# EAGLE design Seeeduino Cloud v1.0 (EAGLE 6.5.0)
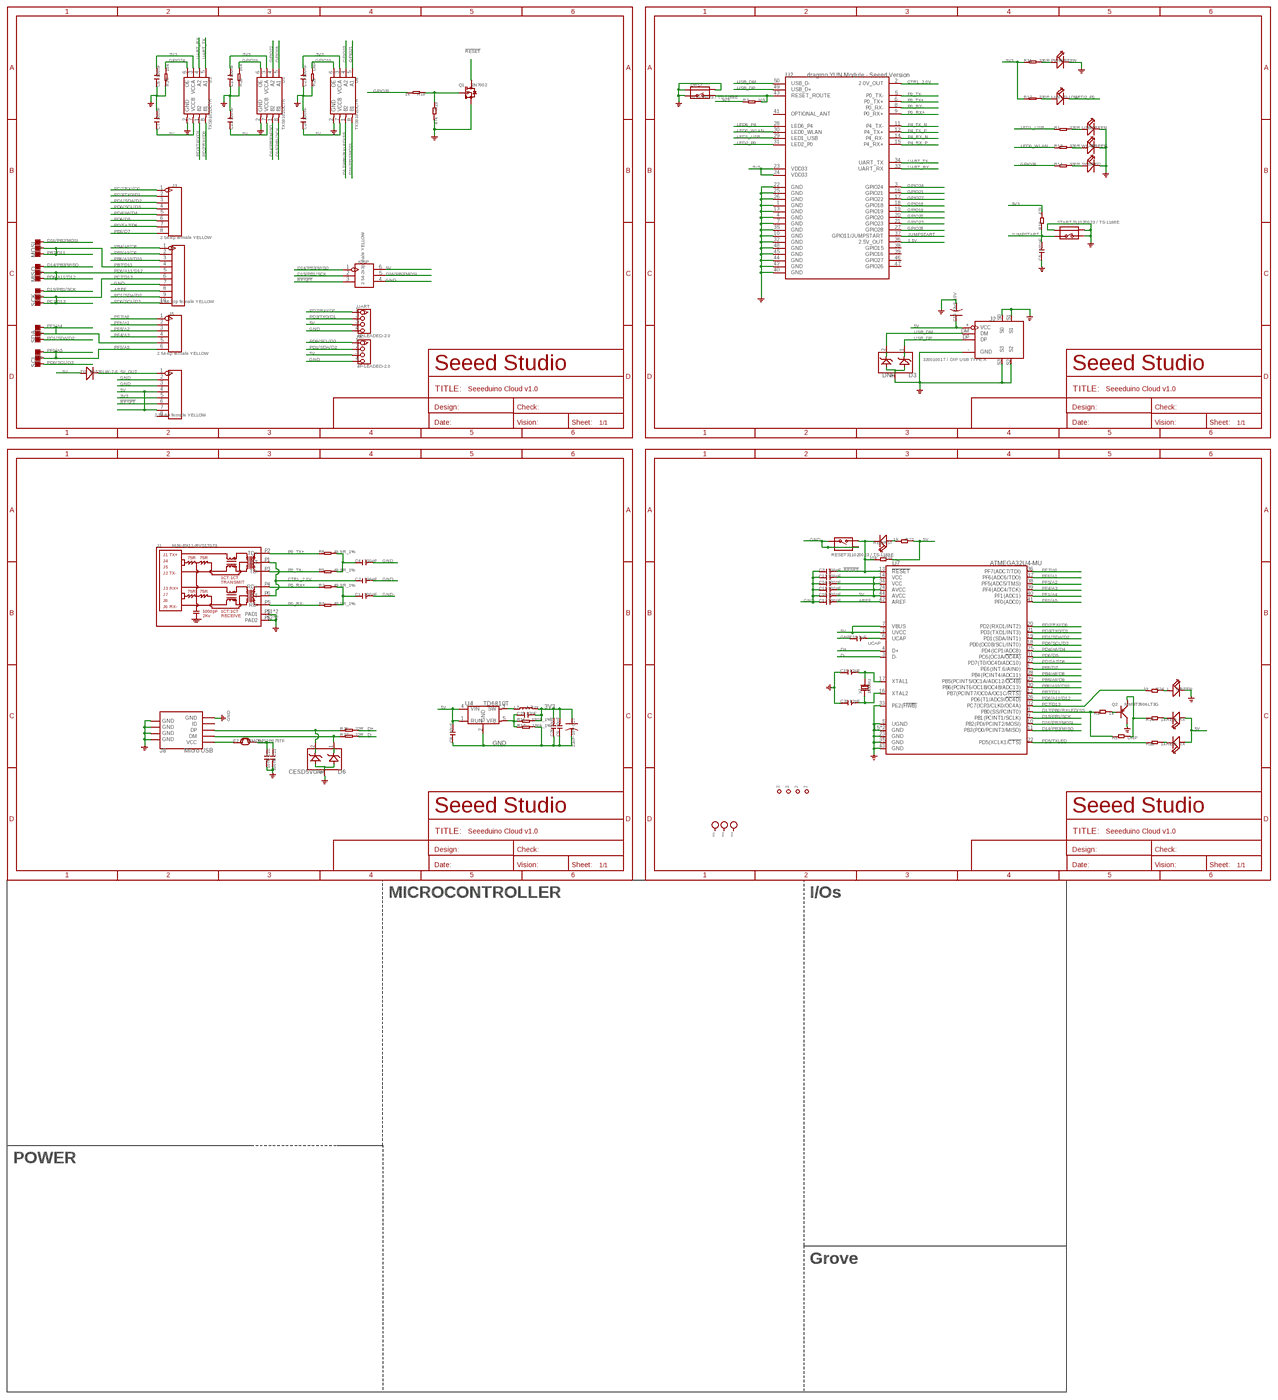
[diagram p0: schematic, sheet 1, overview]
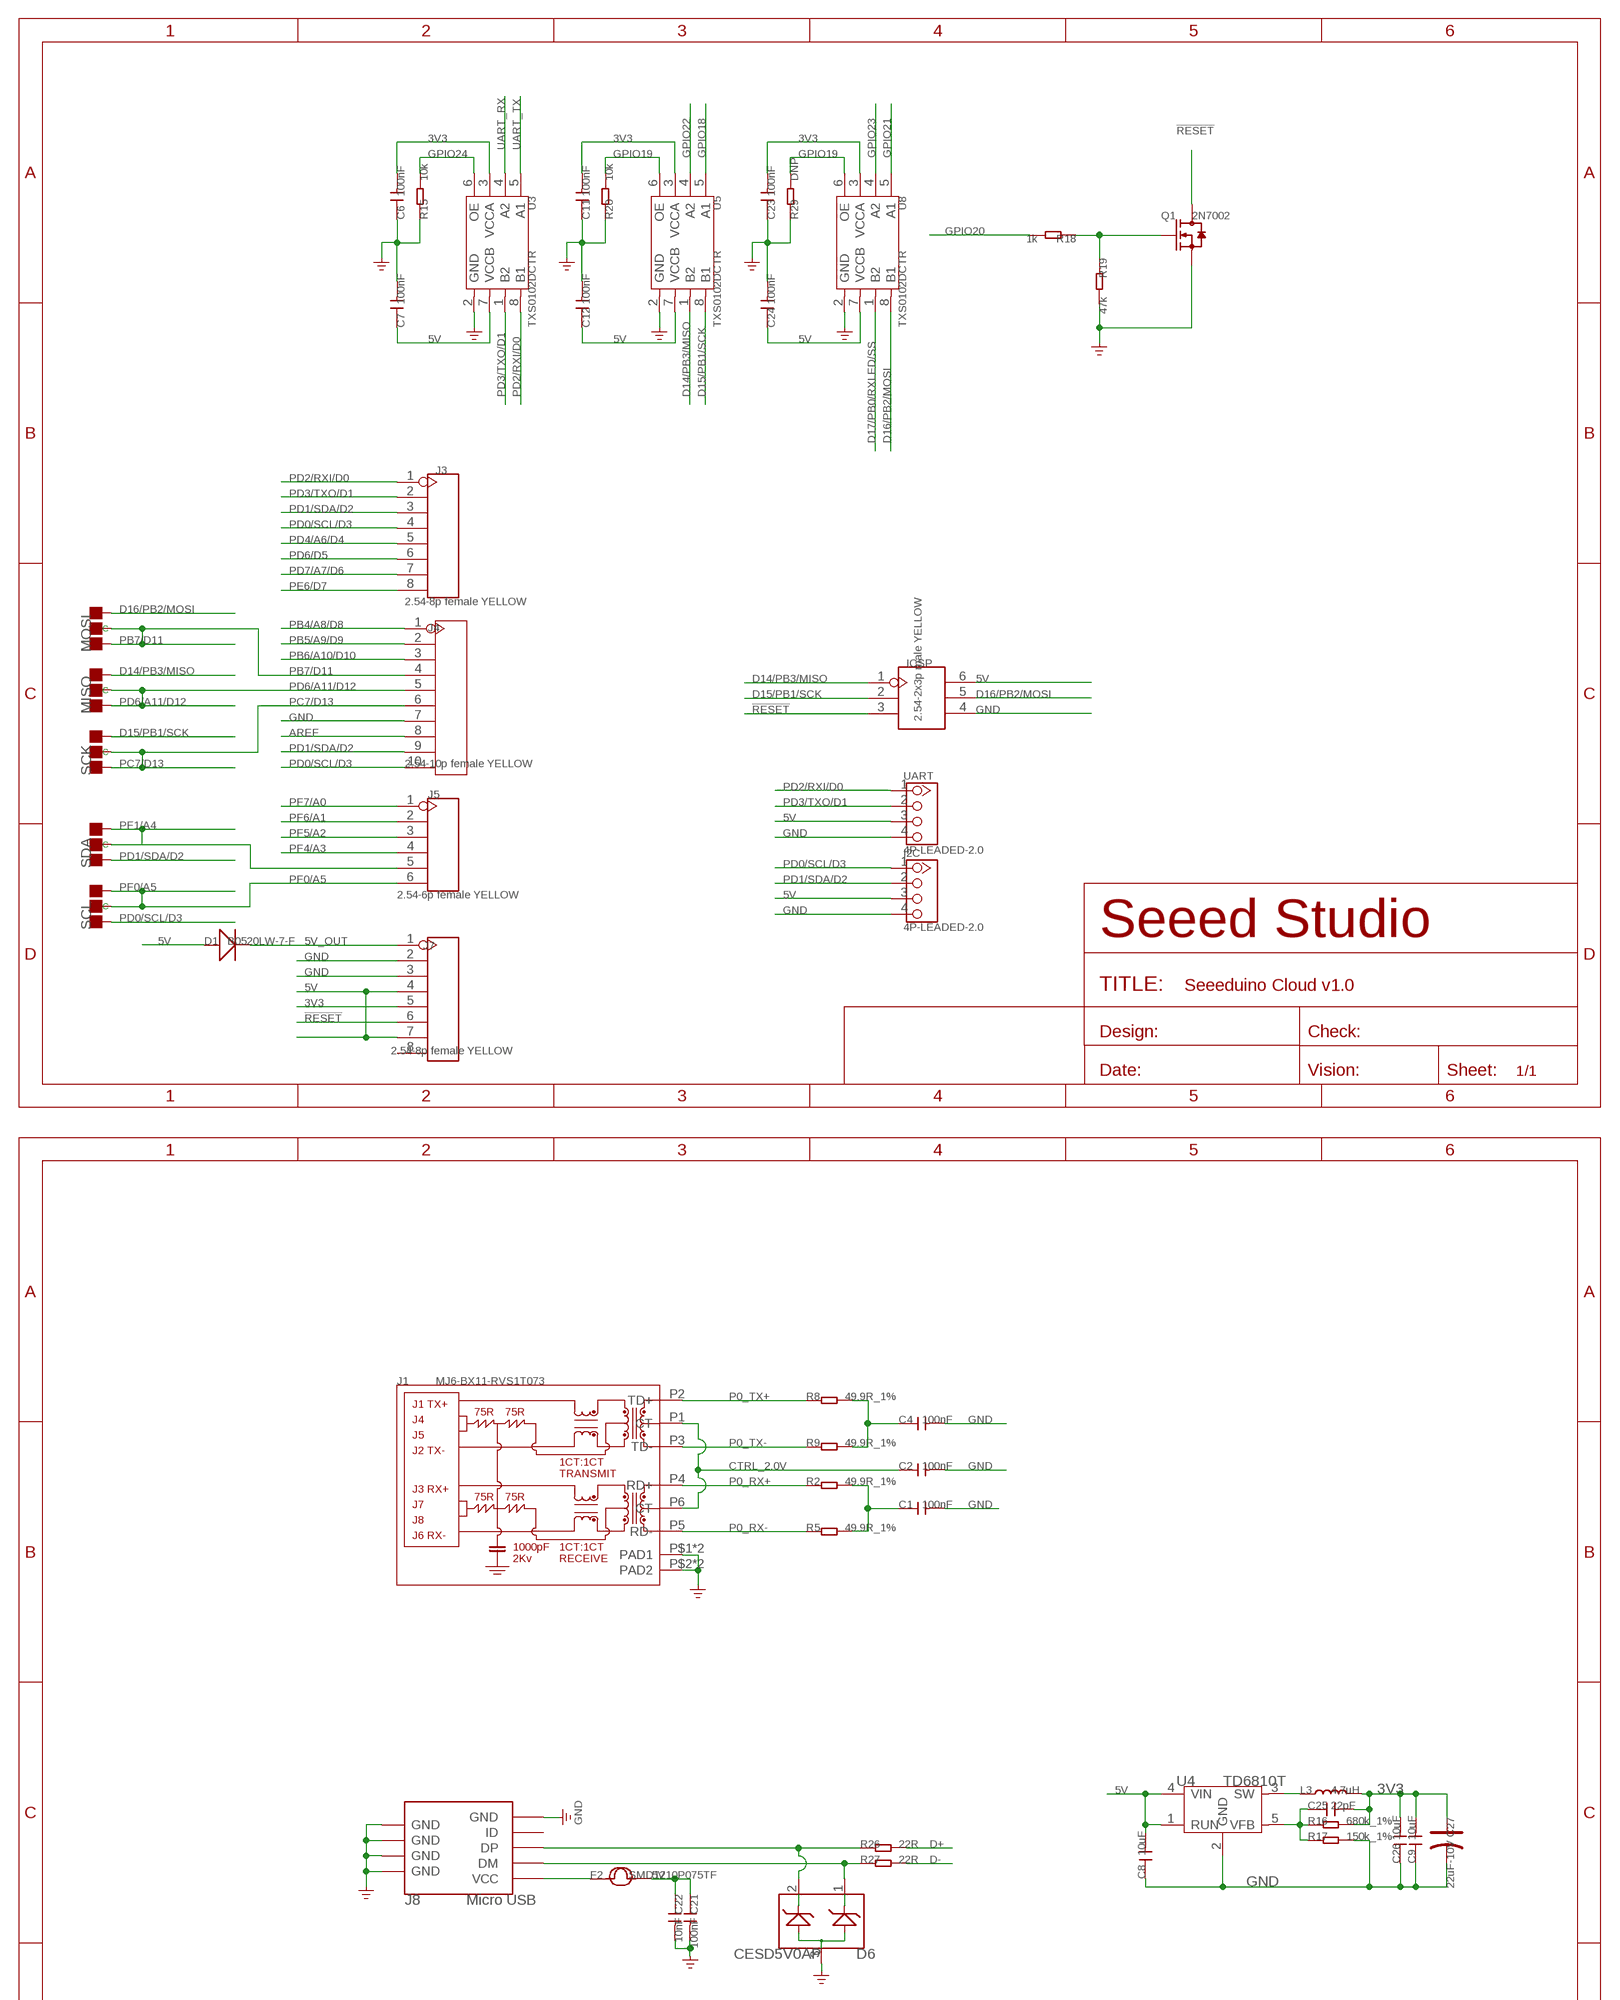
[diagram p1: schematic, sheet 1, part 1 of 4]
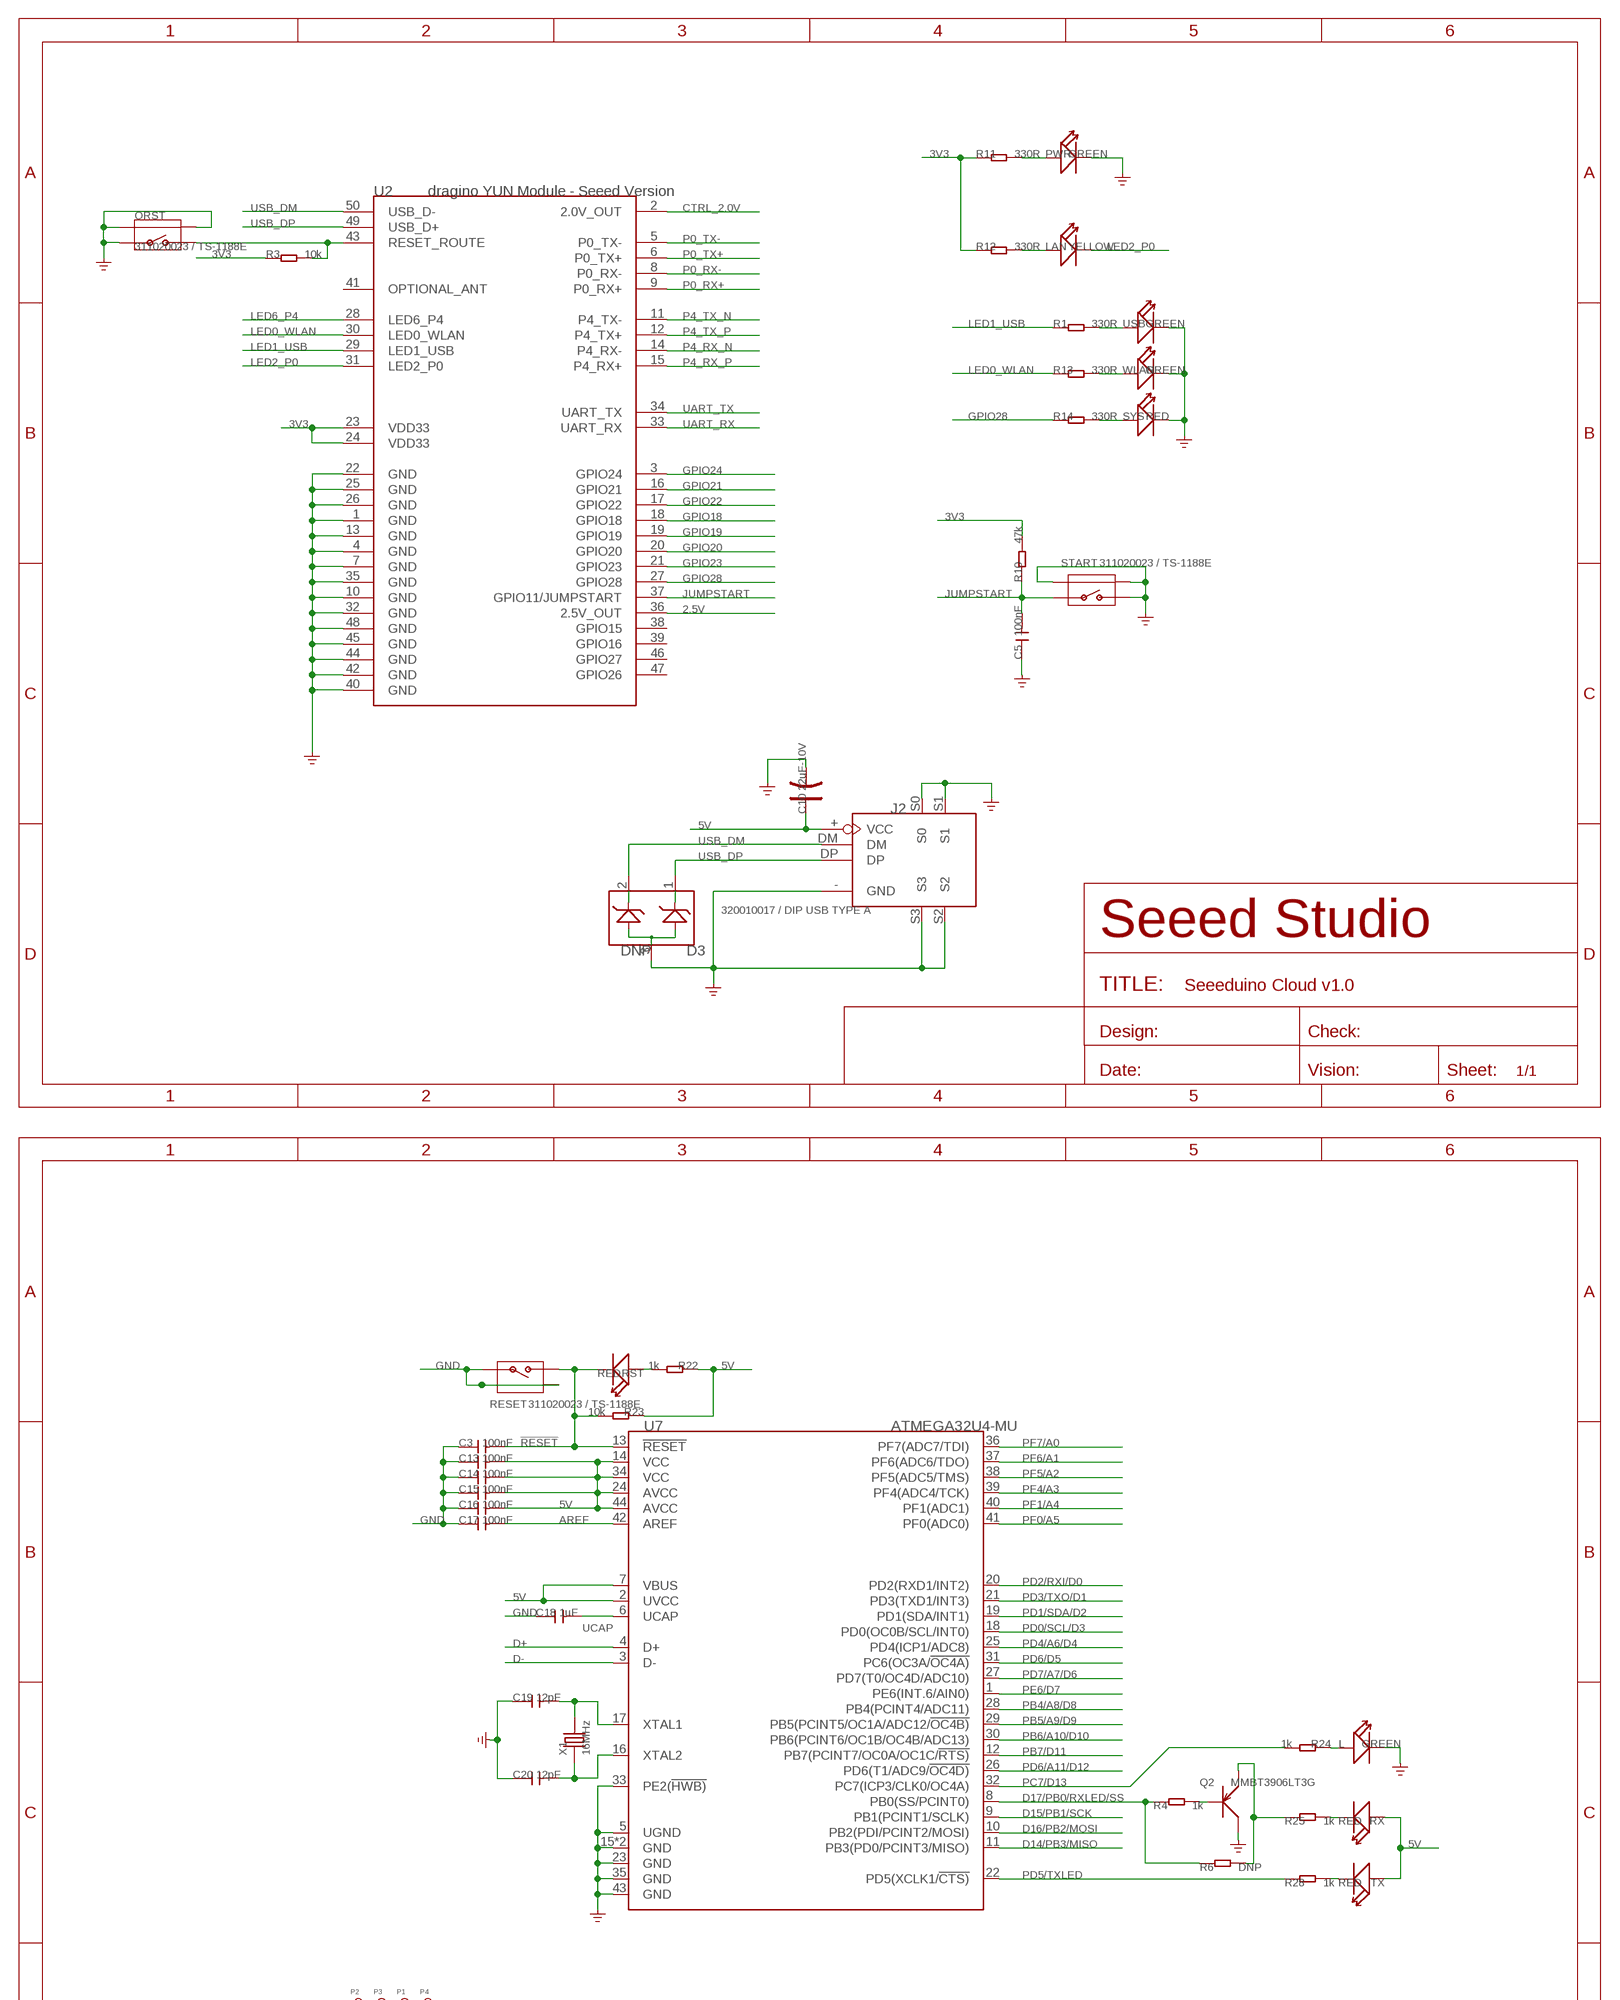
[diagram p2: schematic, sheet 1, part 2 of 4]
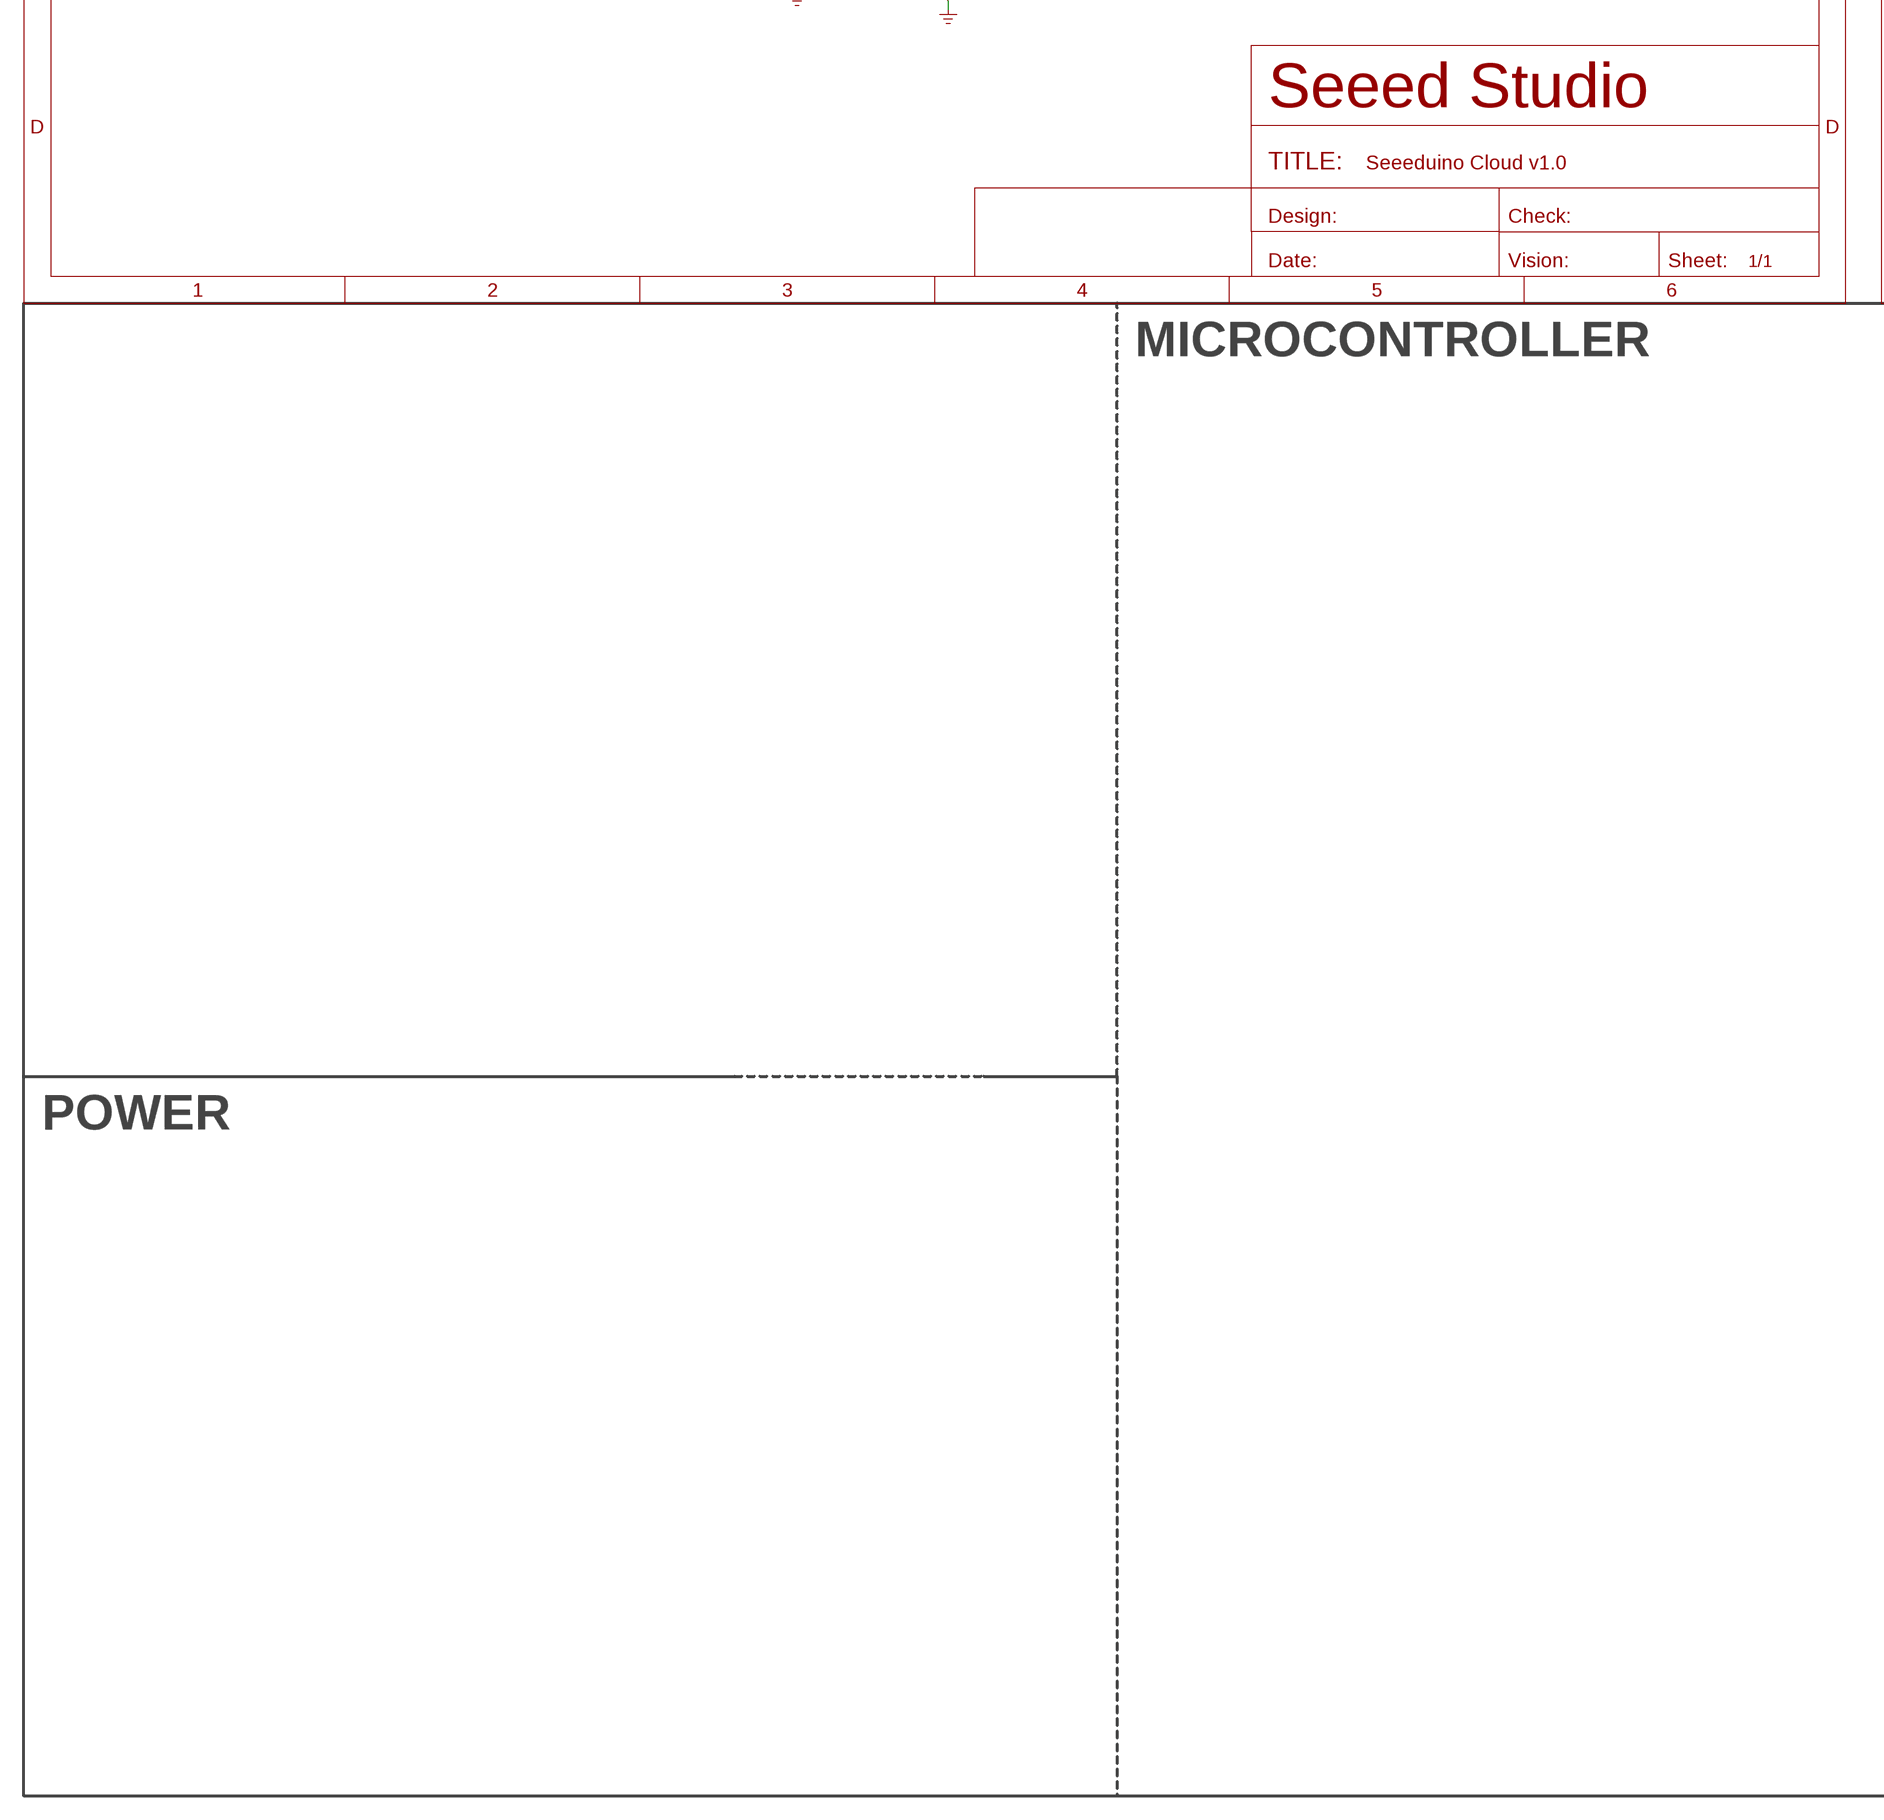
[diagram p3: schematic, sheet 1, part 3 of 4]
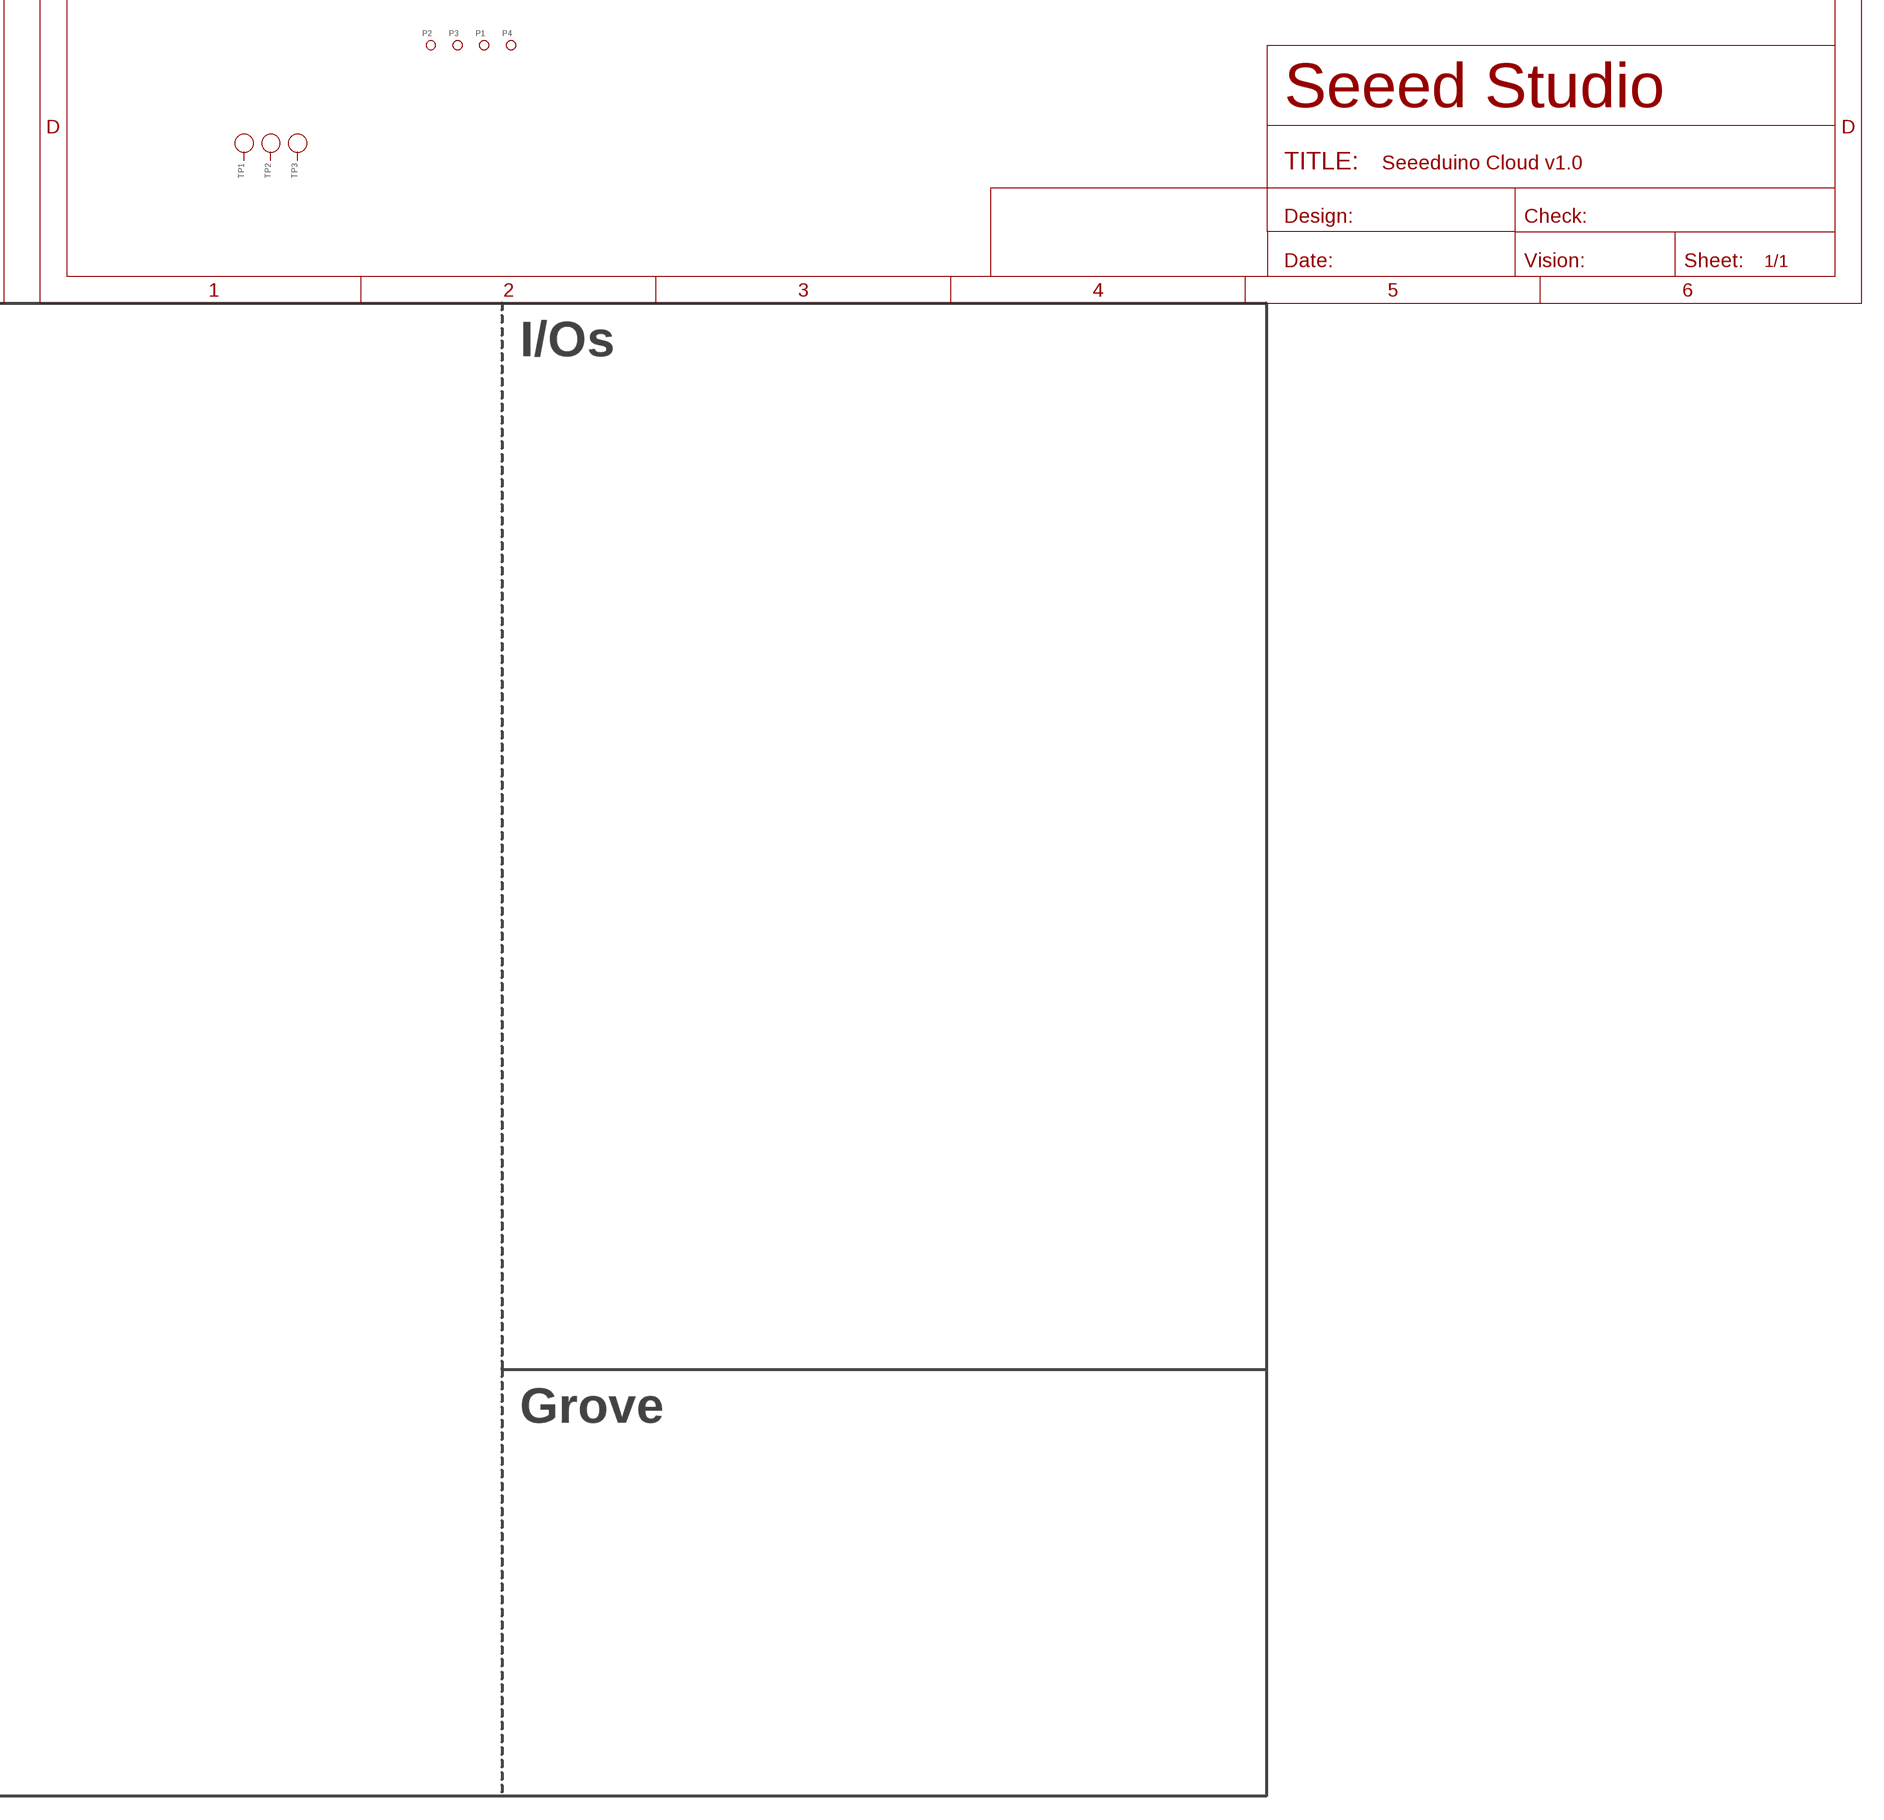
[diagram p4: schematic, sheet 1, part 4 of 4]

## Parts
C1  100nF  C-0402  [C0402]
C2  100nF  C-0402  [C0402]
C3  100nF  C-0402  [C0402]
C4  100nF  C-0402  [C0402]
C5  100nF  C-0402  [C0402]
C6  100nF  C-0402  [C0402]
C7  100nF  C-0402  [C0402]
C8  10uF  C-0805  [C0805]
C9  10uF  C-0805  [C0805]
C10  22uF-10V  CAP-AVX-B  [AVX-B]
C11  100nF  C-0402  [C0402]
C12  100nF  C-0402  [C0402]
C13  100nF  C-0402  [C0402]
C14  100nF  C-0402  [C0402]
C15  100nF  C-0402  [C0402]
C16  100nF  C-0402  [C0402]
C17  100nF  C-0402  [C0402]
C18  1uF  C-0603  [C0603]
C19  12pF  C-0402  [C0402]
C20  12pF  C-0402  [C0402]
C21  100nF  C-0402  [C0402]
C22  10nF  C-0402  [C0402]
C23  100nF  C-0402  [C0402]
C24  100nF  C-0402  [C0402]
C25  22pF  C-0603  [C0603]
C26  10uF  C-0805  [C0805]
C27  22uF-10V  CAP-AVX-B  [AVX-B]
D1  B0520LW-7-F  D'1206'  [SOD123]
D3  DNP  D-ESD-3P  [SOT23]
D6  CESD5V0AP  D-ESD-3P  [SOT23]
F2  SMD1210P075TF  FUSE'1206'  [F1206]
I2C  4P-LEADED-2.0  TWIG-2.0-LEADED  [4P-LEADED-2.0]
ICSP  2.54-2x3p male YELLOW  HEADER-2X3P-2.54  [2X3P-2.54]
J1  MJ6-BX11-RVS1T073  CONNECTOR-RJ45+TRAMSFORMER-MJ6-BX11-RVS1T073  [RJ45-MJ6-BX11-RVS1T073]
J2  320010017 / DIP USB TYPE A  USB-FEMALE-13.2X14.5  [FEMALE-14.5X13.2]
J3  2.54-8p female YELLOW  HEADER-8P-65/35MIL  [8P-2.54-65/35MIL]
J4  2.54-10p female YELLOW  HEADER-10P-2.54  [10P-2.54]
J5  2.54-6p female YELLOW  HEADER-6P-65/35MIL  [6P-2.54-65/35MIL]
J7  2.54-8p female YELLOW  HEADER-8P-65/35MIL  [8P-2.54-65/35MIL]
J8  Micro USB  USB-MINIUSB-5P-MICRO  [MICRO-USB]
L  GREEN  LED-0603  [LED-0603]
L3  4.7uH  L-04XX  [04XX]
LAN  YELLOW  LED-0603  [LED-0603]
MISO  DNP  PAD-JUMPER-3P-40*40  [3P-SMD-4.1X1.5]
MOSI  DNP  PAD-JUMPER-3P-40*40  [3P-SMD-4.1X1.5]
ORST  311020023 / TS-1188E  BUTTON-4P-REINFORCE'TS-1188E'  [4P-SMD-7X3.5X3.5H]
P1  PAD-MARK'ANNULAR'  [ROUND-MARK-1.0]
P2  PAD-MARK'ANNULAR'  [ROUND-MARK-1.0]
P3  PAD-MARK'ANNULAR'  [ROUND-MARK-1.0]
P4  PAD-MARK'ANNULAR'  [ROUND-MARK-1.0]
PWR  GREEN  LED-0603  [LED-0603]
Q1  2N7002  MOSFET-N'SOT23'  [SOT23]
Q2  MMBT3906LT3G  TRANSISTOR-PNP-SOT23  [SOT23]
R1  330R  R-0402  [R0402]
R2  49.9R_1%  R-0402  [R0402]
R3  10k  R-0402  [R0402]
R4  1k  R-0402  [R0402]
R5  49.9R_1%  R-0402  [R0402]
R6  DNP  R-0402  [R0402]
R8  49.9R_1%  R-0402  [R0402]
R9  49.9R_1%  R-0402  [R0402]
R10  47k  R-0402  [R0402]
R11  330R  R-0402  [R0402]
R12  330R  R-0402  [R0402]
R13  330R  R-0402  [R0402]
R14  330R  R-0402  [R0402]
R15  10k  R-0402  [R0402]
R16  680k_1%  R-0603  [R0603]
R17  150k_1%  R-0603  [R0603]
R18  1k  R-0402  [R0402]
R19  47k  R-0402  [R0402]
R20  10k  R-0402  [R0402]
R22  1k  R-0402  [R0402]
R23  10k  R-0402  [R0402]
R24  1k  R-0402  [R0402]
R25  1k  R-0402  [R0402]
R26  22R  R-0402  [R0402]
R27  22R  R-0402  [R0402]
R28  1k  R-0402  [R0402]
R29  DNP  R-0402  [R0402]
RESET  311020023 / TS-1188E  BUTTON-4P-REINFORCE'TS-1188E'  [4P-SMD-7X3.5X3.5H]
RST  RED  LED-0603  [LED-0603]
RX  RED  LED-0603  [LED-0603]
SCK  DNP  PAD-JUMPER-3P-40*40  [3P-SMD-4.1X1.5]
SCL  DNP  PAD-JUMPER-3P-40*40  [3P-SMD-4.1X1.5]
SDA  DNP  PAD-JUMPER-3P-40*40  [3P-SMD-4.1X1.5]
START  311020023 / TS-1188E  BUTTON-4P-REINFORCE'TS-1188E'  [4P-SMD-7X3.5X3.5H]
SYS  RED  LED-0603  [LED-0603]
TP1  DNP  PAD-TEST-POINT'4545'  [TP_4545]
TP2  DNP  PAD-TEST-POINT'4545'  [TP_4545]
TP3  DNP  PAD-TEST-POINT'4545'  [TP_4545]
TX  RED  LED-0603  [LED-0603]
U2  dragino YUN Module - Seeed Version  HE  [HE50]
U3  TXS0102DCTR  TXS0102-DCT  [PDSO-G8]
U4  TD6810T  TD6810'TSOT23-5'  [SOT23-5]
U5  TXS0102DCTR  TXS0102-DCT  [PDSO-G8]
U7  ATMEGA32U4-MU  [QFN44]
U8  TXS0102DCTR  TXS0102-DCT  [PDSO-G8]
UART  4P-LEADED-2.0  TWIG-2.0-LEADED  [4P-LEADED-2.0]
USB  GREEN  LED-0603  [LED-0603]
WLAN  GREEN  LED-0603  [LED-0603]
X1  16MHz  CRYSTAL'5032'  [2P-SMD-5X3.2]

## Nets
2.5V: U2.36(2.5V_OUT)
3V3: C6.2 C9.2 C11.2 C23.2 C25.2 C26.2 C27.+ J7.5 L3.2 R3.1 R10.2 R11.1 R12.1 R16.2 U2.23(VDD33) U2.24(VDD33) U3.3(VCCA) U5.3(VCCA) U8.3(VCCA)
5V: C7.1 C8.2 C10.+ C12.1 C13.2 C14.2 C15.2 C16.2 C21.1 C22.1 C24.1 D1.+ F2.2 I2C.3 ICSP.6 J2.+(VCC) J7.4 J7.7 R22.1 R23.1 RX.+ TX.+ U3.7(VCCB) U4.1(RUN) U4.4(VIN) U5.7(VCCB) U7.2(UVCC) U7.7(VBUS) U7.14(VCC) U7.24(AVCC) U7.34(VCC) U7.44(AVCC) U8.7(VCCB) UART.3
5V_OUT: D1.- J7.1
!RESET: C3.2 ICSP.3 J7.6 Q1.3(D) R23.2 RESET.2 RST.- U7.13(!RESET)
AREF: C17.2 J4.8 U7.42(AREF)
CTRL_2.0V: C2.1 J1.P1(CT) J1.P6(CT) U2.2(2.0V_OUT)
D14/PB3/MISO: ICSP.1 MISO.00(L) U5.1(B2) U7.11(PB3(PD0/PCINT3/MISO))
D15/PB1/SCK: ICSP.2 SCK.00(L) U5.8(B1) U7.9(PB1(PCINT1/SCLK))
D16/PB2/MOSI: ICSP.5 MOSI.00(L) U7.10(PB2(PDI/PCINT2/MOSI)) U8.8(B1)
D17/PB0/RXLED/SS: R4.1 R6.1 U7.8(PB0(SS/PCINT0)) U8.1(B2)
D+: R26.2 U7.4(D+)
D-: R27.2 U7.3(D-)
GND: C1.2 C2.2 C3.1 C4.2 C5.1 C6.1 C7.2 C8.1 C9.1 C10.- C11.1 C12.2 C13.1 C14.1 C15.1 C16.1 C17.1 C18.1 C19.1 C20.1 C21.2 C22.2 C23.1 C24.2 C26.1 C27.- D3.3 D6.3 I2C.4 ICSP.4 J1.P$1(PAD1) J1.P$2(PAD2) J1.PAD1 J1.PAD2 J2.-(GND) J2.S0 J2.S1 J2.S2 J2.S3 J4.7 J7.2 J7.3 J8.5(GND) J8.S1(GND) J8.S2(GND) J8.S3(GND) J8.S4(GND) J8.S5(GND) J8.S6(GND) L.- ORST.1 ORST.S1 ORST.S2 PWR.- Q1.2(S) Q2.3(C) R15.1 R17.2 R19.2 R20.1 R29.1 RESET.1 RESET.S1 RESET.S2 START.2 START.S1 START.S2 SYS.- U2.1(GND) U2.4(GND) U2.7(GND) U2.10(GND) U2.13(GND) U2.22(GND) U2.25(GND) U2.26(GND) U2.32(GND) U2.35(GND) U2.40(GND) U2.42(GND) U2.44(GND) U2.45(GND) U2.48(GND) U3.2(GND) U4.2(GND) U5.2(GND) U7.5(UGND) U7.15(GND) U7.23(GND) U7.33(PE2(!HWB)) U7.35(GND) U7.43(GND) U7.TAB(GND) U8.2(GND) UART.4 USB.- WLAN.-
GPIO18: U2.18(GPIO18) U5.5(A1)
GPIO19: R20.2 R29.2 U2.19(GPIO19) U5.6(OE) U8.6(OE)
GPIO20: R18.2 U2.20(GPIO20)
GPIO21: U2.16(GPIO21) U8.5(A1)
GPIO22: U2.17(GPIO22) U5.4(A2)
GPIO23: U2.21(GPIO23) U8.4(A2)
GPIO24: R15.2 U2.3(GPIO24) U3.6(OE)
GPIO28: R14.1 U2.27(GPIO28)
JUMPSTART: C5.2 R10.1 START.1 U2.37(GPIO11/JUMPSTART)
LED0_WLAN: R13.1 U2.30(LED0_WLAN)
LED1_USB: R1.1 U2.29(LED1_USB)
LED2_P0: LAN.- U2.31(LED2_P0)
LED6_P4: U2.28(LED6_P4)
N$1: C19.2 U7.17(XTAL1) X1.2
N$2: C20.2 U7.16(XTAL2) X1.1
N$4: L.+ R24.1
N$5: R28.2 TX.-
N$6: D6.1 J8.2(DM) R27.1
N$7: Q2.2(E) R6.2 R25.1
N$8: D6.2 J8.3(DP) R26.1
N$9: L3.1 U4.3(SW)
N$10: R1.2 USB.+
N$11: C25.1 R16.1 R17.1 U4.5(VFB)
N$12: F2.1 J8.1(VCC)
N$13: Q1.1(G) R18.1 R19.1
N$14: C1.1 R2.2 R5.2
N$15: ORST.2 R3.2 U2.43(RESET_ROUTE)
N$16: R25.2 RX.-
N$17: R22.2 RST.+
N$18: C4.1 R8.2 R9.2
N$19: Q2.1(B) R4.2
N$23: PWR.+ R11.2
N$24: LAN.+ R12.2
N$25: R13.2 WLAN.+
N$26: R14.2 SYS.+
P0_RX+: J1.P4(RD+) R2.1 U2.9(P0_RX+)
P0_RX-: J1.P5(RD-) R5.1 U2.8(P0_RX-)
P0_TX+: J1.P2(TD+) R8.1 U2.6(P0_TX+)
P0_TX-: J1.P3(TD-) R9.1 U2.5(P0_TX-)
P4_RX_N: U2.14(P4_RX-)
P4_RX_P: U2.15(P4_RX+)
P4_TX_N: U2.11(P4_TX-)
P4_TX_P: U2.12(P4_TX+)
PB4/A8/D8: J4.1 U7.28(PB4(PCINT4/ADC11))
PB5/A9/D9: J4.2 U7.29(PB5(PCINT5/OC1A/ADC12/!OC4B))
PB6/A10/D10: J4.3 U7.30(PB6(PCINT6/OC1B/OC4B/ADC13))
PB7/D11: J4.4 MOSI.11(R) MOSI.MM(C) U7.12(PB7(PCINT7/OC0A/OC1C/!RTS))
PC7/D13: J4.6 R24.2 SCK.11(R) SCK.MM(C) U7.32(PC7(ICP3/CLK0/OC4A))
PD0/SCL/D3: I2C.1 J3.4 J4.10 SCL.11(R) U7.18(PD0(OC0B/SCL/INT0))
PD1/SDA/D2: I2C.2 J3.3 J4.9 SDA.11(R) U7.19(PD1(SDA/INT1))
PD2/RXI/D0: J3.1 U3.8(B1) U7.20(PD2(RXD1/INT2)) UART.1
PD3/TXO/D1: J3.2 U3.1(B2) U7.21(PD3(TXD1/INT3)) UART.2
PD4/A6/D4: J3.5 U7.25(PD4(ICP1/ADC8))
PD5/TXLED: R28.1 U7.22(PD5(XCLK1/!CTS))
PD6/A11/D12: J4.5 MISO.11(R) MISO.MM(C) U7.26(PD6(T1/ADC9/!OC4D))
PD6/D5: J3.6 U7.31(PC6(OC3A/!OC4A))
PD7/A7/D6: J3.7 U7.27(PD7(T0/OC4D/ADC10))
PE6/D7: J3.8 U7.1(PE6(INT.6/AIN0))
PF0/A5: J5.6 SCL.00(L) SCL.MM(C) U7.41(PF0(ADC0))
PF1/A4: J5.5 SDA.00(L) SDA.MM(C) U7.40(PF1(ADC1))
PF4/A3: J5.4 U7.39(PF4(ADC4/TCK))
PF5/A2: J5.3 U7.38(PF5(ADC5/TMS))
PF6/A1: J5.2 U7.37(PF6(ADC6/TDO))
PF7/A0: J5.1 U7.36(PF7(ADC7/TDI))
UART_RX: U2.33(UART_RX) U3.4(A2)
UART_TX: U2.34(UART_TX) U3.5(A1)
UCAP: C18.2 U7.6(UCAP)
USB_DM: D3.2 J2.DM U2.50(USB_D-)
USB_DP: D3.1 J2.DP U2.49(USB_D+)
Unconnected: J7.8 J8.4(ID) TP1.T TP2.T TP3.T U2.38(GPIO15) U2.39(GPIO16) U2.46(GPIO27) U2.47(GPIO26)

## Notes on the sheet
- MICROCONTROLLER | I/Os
- POWER
- Grove

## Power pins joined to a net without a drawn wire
OPTIONAL_ANT: U2.41(OPTIONAL_ANT)

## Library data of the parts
C1-C9 C11-C26 = Discrete:C*: Ceramic Capacitors
C10 C27 = Discrete:CAP*: Electrolytic Capacitors,Tantalum Capacitors and Super Capacitors
D1 = Discrete:D*
D3 D6 = Discrete:D-ESD-3P
F2 = Discrete:FUSE
I2C UART = Connector:TWIG-2.0-LEADED
ICSP = Connector:HEADER-2X3P
J1 = template:CONNECTOR-RJ45+TRAMSFORMER-MJ6-BX11-RVS1T073: RJ45+Transformer
J2 = Connector:USB-FEMALE
J3 J7 = Connector:HEADER-8P
J4 = Connector:HEADER-10P
J5 = Connector:HEADER-6P
J8 = Connector:USB-MINIUSB-5P
L LAN PWR RST RX SYS TX USB WLAN = AMLib_New:LED
L3 = Sata:L*
MISO MOSI SCK SCL SDA = Discrete:PAD-JUMPER-3P; PARTNO: DNP
ORST RESET START = Discrete:BUTTON-4P-REINFORCE: TS-1188E http://www.best-dz.com/?thread-374-2.html
P1-P4 = Discrete:PAD-MARK; PARTNO: DNP
Q1 = Discrete:MOSFET-N: IRLL014: http://www.vishay.com/docs/91319/sihll014.pdf
Q2 = Discrete:TRANSISTOR-PNP*: PNP audion
R1-R6 R8-R20 R22-R29 = Discrete:R*
TP1-TP3 = Discrete:PAD-TEST-POINT; PARTNO: DNP
U2 = dragino:HE
U3 U5 U8 = AMLib_New:TXS0102
U4 = template:TD6810: 1.5MHz 800mA Synchronous Step-Down Regulator Dropout http://www.techcodeok.com/download/TD6810.pdf
U7 = IC:ATMEGA32U4: 8-bit Microcontroller With 16/32K Bytes of ISP Flash and USB controller
X1 = Discrete:CRYSTAL*: CRYSTAL

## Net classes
0 default: width 0.152 mm, drill 0.305 mm, clearance 0.152 mm

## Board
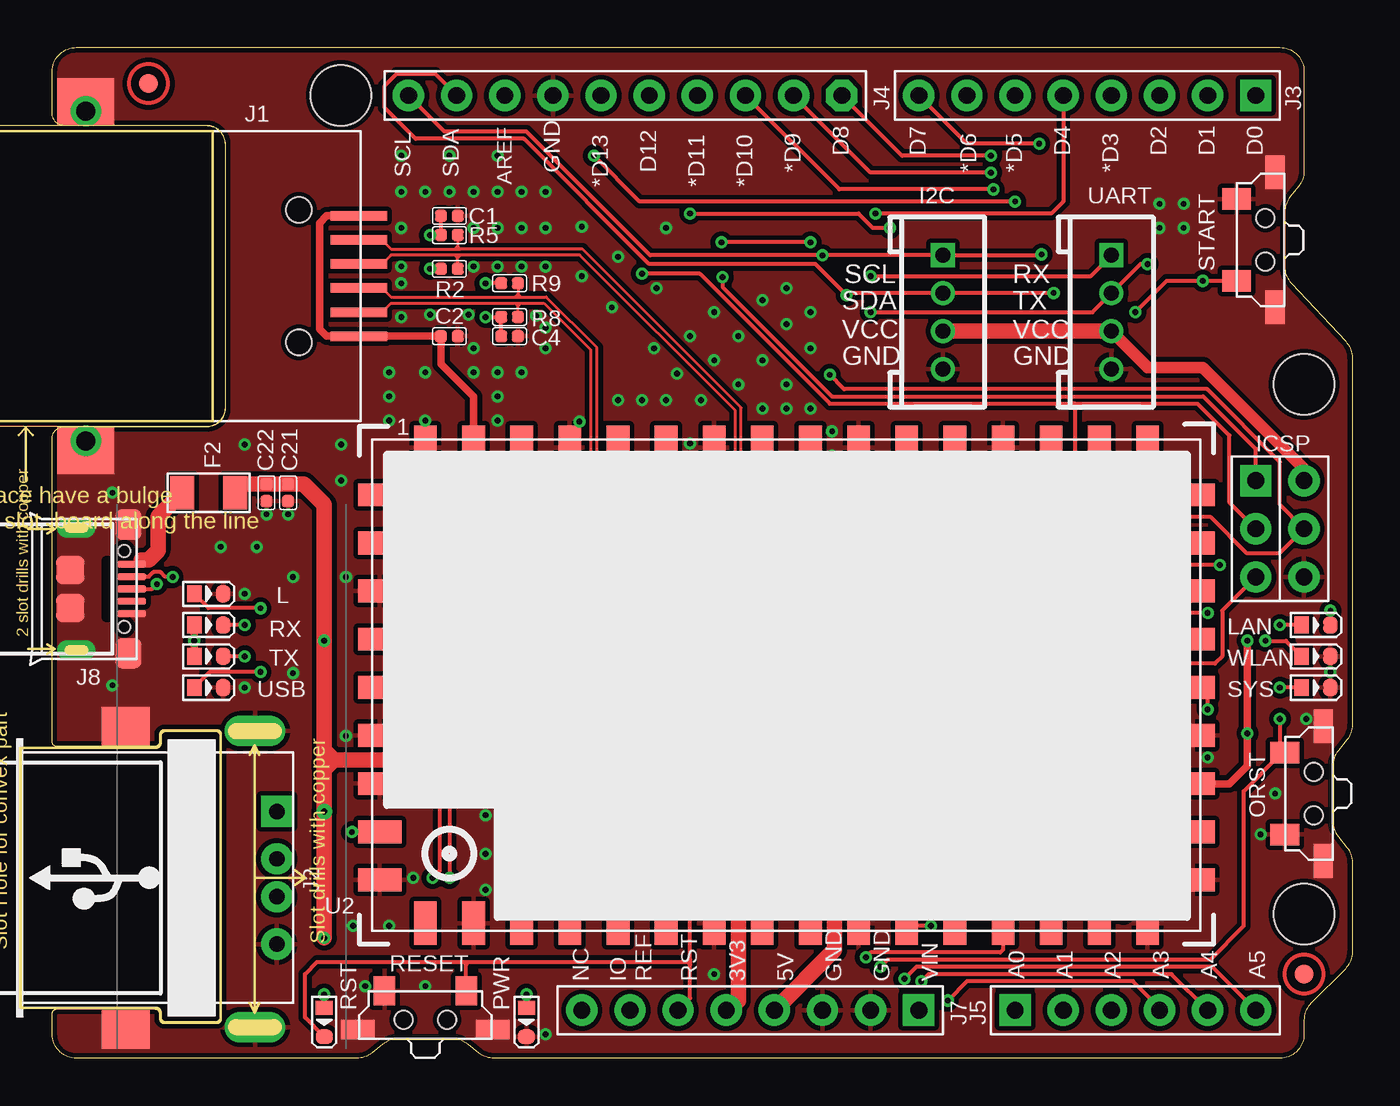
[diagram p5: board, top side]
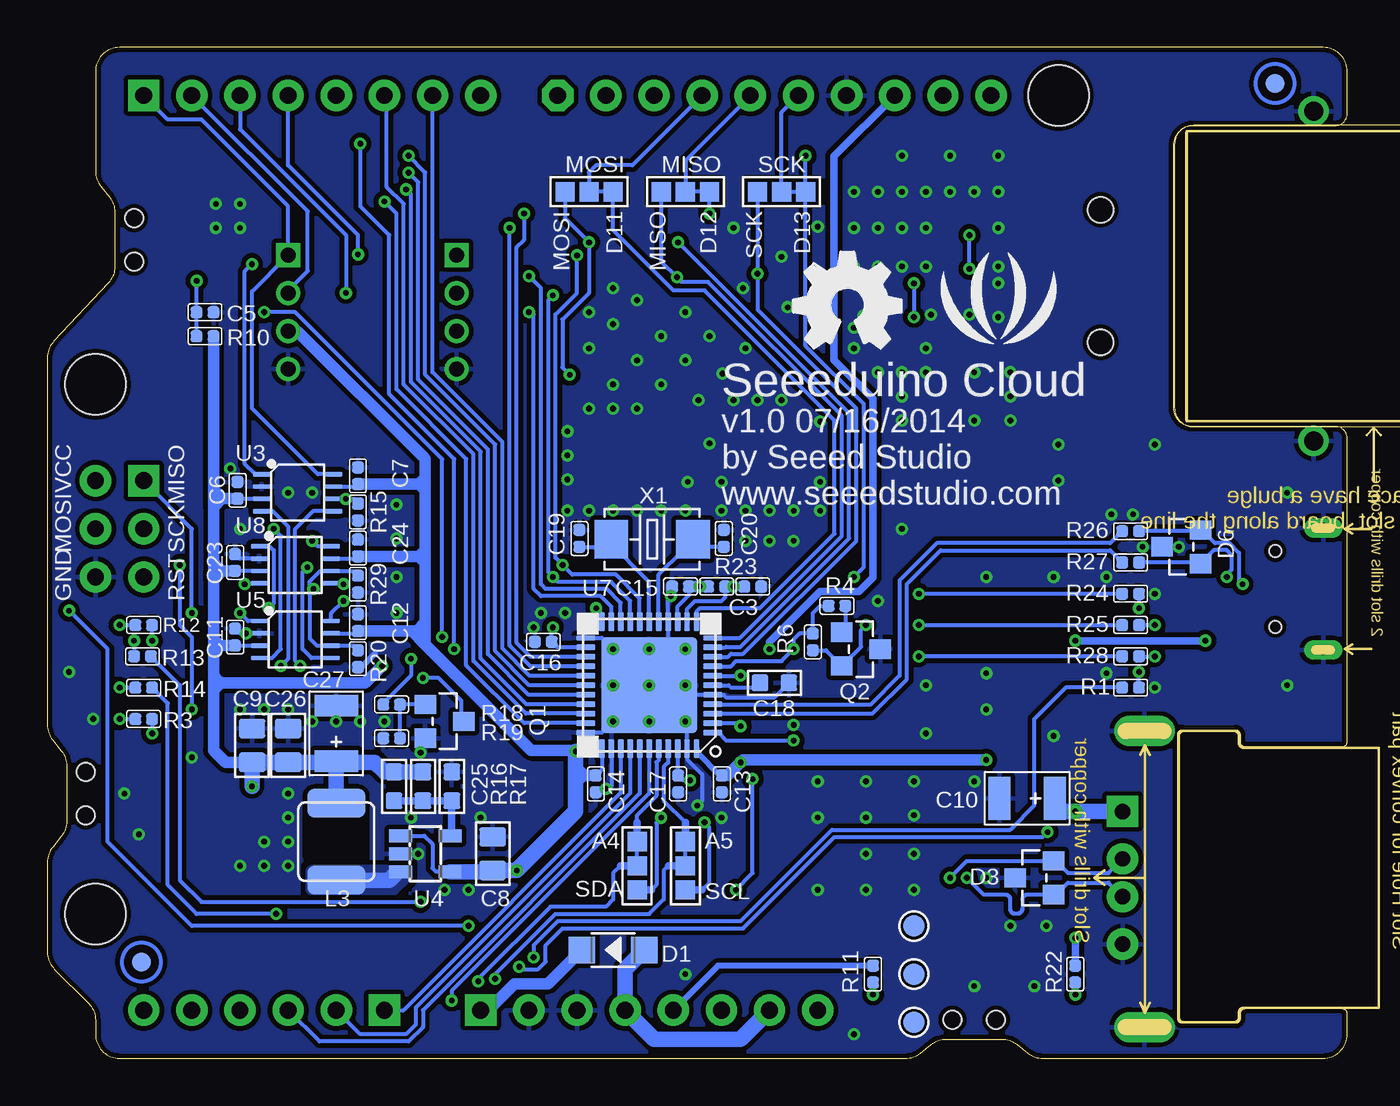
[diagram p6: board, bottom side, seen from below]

Size 68.58 x 53.34 mm. Coordinates in mm from the lower left corner, seen from the top.
Outline: 60 segments
Copper layers (1*16): Top 0.035mm / dielectric 1.5mm / Bottom 0.035mm
Design rules "SeeedStudio_rule_no_angle_090911 *": minimum track width 6mil, minimum drill 12mil, track to track 6mil, track to pad 6mil, pad to pad 6mil, via to via 6mil, smd to smd 0mil, copper to edge 10mil, drill to drill 10mil, minimum pad ring 8mil, minimum via ring 6mil, stop-mask expansion 2mil, vias tented up to drill 25mil, thermal gap 10mil
Holes 3.2 mm at 15.24,50.8 66.04,35.56 66.04,7.62
bRestrict: area 51.8,10.7 to 54.9,13.7

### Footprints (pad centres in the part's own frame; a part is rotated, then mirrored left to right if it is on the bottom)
C0402 = smd 0.635 x 0.635: 1 -0.445,0; 2 0.445,0
C0805 = smd 1.016 x 1.397: 1 -0.889,0; 2 0.889,0
AVX-B = smd 1.143 x 2.286: + -1.46,0; - 1.46,0
C0603 = smd 0.889 x 0.889: 1 -0.762,0; 2 0.762,0
SOD123 = smd 1.397 x 1.397: + -1.651,0; - 1.651,0
SOT23 = smd 1.016 x 1.143: 1 -0.889,-1.016; 2 0.889,-1.016; 3 0,1.016
F1206 = smd 1.27 x 1.778: 1 -1.397,0; 2 1.397,0
4P-LEADED-2.0 = drill 0.8 pad 1.27 square: 1 -3,0 | drill 0.8 pad 1.27: 2 -1,0; 3 1,0; 4 3,0
2X3P-2.54 = drill 0.889 pad 1.651 square: 1 -1.27,2.54 | drill 0.889 pad 1.651: 2 -1.27,0; 3 -1.27,-2.54; 4 1.27,-2.54; 5 1.27,0; 6 1.27,2.54
RJ45-MJ6-BX11-RVS1T073 = smd 0.5 x 3: P1 3.175,14.4; P2 1.905,14.4; P3 0.635,14.4; P4 -0.635,14.4; P5 -1.905,14.4; P6 -3.175,14.4 | smd 2.5 x 3: P$1 -9.2,0; P$2 9.2,0 | drill 1 pad 1.6: PAD1 -8.7,0; PAD2 8.7,0 | hole 1.35: -3.5,11.24; 3.5,11.24
FEMALE-14.5X13.2 = drill 0.813 pad 1.651 square: + 0.85,-3.5 | drill 0.813 pad 1.651: - 0.85,3.5; DM 0.85,-1; DP 0.85,1 | smd 2.54 x 2.032: S0 8.83,8.001; S3 8.83,-8.001 | drill 0.7 pad 1.6 long: S1 2,7.874; S2 2,-7.747
8P-2.54-65/35MIL = drill 0.889 pad 1.651 square: 1 0,8.89 | drill 0.889 pad 1.651: 2 0,6.35; 3 0,3.81; 4 0,1.27; 5 0,-1.27; 6 0,-3.81; 7 0,-6.35; 8 0,-8.89
10P-2.54 = drill 0.889 pad 1.651 octagon: 1 0,11.43 | drill 0.889 pad 1.651: 2 0,8.89; 3 0,6.35; 4 0,3.81; 5 0,1.27; 6 0,-1.27; 7 0,-3.81; 8 0,-6.35; 9 0,-8.89; 10 0,-11.43
6P-2.54-65/35MIL = drill 0.889 pad 1.651 square: 1 0,6.35 | drill 0.889 pad 1.651: 2 0,3.81; 3 0,1.27; 4 0,-1.27; 5 0,-3.81; 6 0,-6.35
MICRO-USB = smd 0.381 x 1.524: 1 -1.3,-0.25; 2 -0.65,-0.25; 3 0,-0.25; 4 0.65,-0.25; 5 1.3,-0.25 | smd 1.6 x 1.397: S1 -3.4,-0.427; S6 3.4,-0.427 | drill 0.508 pad 1.016 long: S2 -3.226,-3.175; S5 3.226,-3.175 | smd 1.5 x 1.5: S3 -1,-3.5; S4 1,-3.5 | hole 0.635: -2,-0.65; 2,-0.65
LED-0603 = smd 0.762 x 0.889: + -0.762,0; - 0.762,0
04XX = smd 1.524 x 3.048: 1 -2.032,0; 2 2.032,0
3P-SMD-4.1X1.5 = smd 1.016 x 1.016: 00 -1.27,0; 11 1.27,0; MM 0,0
4P-SMD-7X3.5X3.5H = smd 1.143 x 1.524: 1 -2.159,1.524; 2 2.159,1.524 | smd 1.778 x 1.016: S1 -3.556,-0.508; S2 3.556,-0.508 | hole 0.95: -1.15,0; 1.15,0
ROUND-MARK-1.0 = smd 1.016 x 1.016: P$1 0,0
R0402 = smd 0.635 x 0.635: 1 -0.445,0; 2 0.445,0
R0603 = smd 0.889 x 0.889: 1 -0.762,0; 2 0.762,0
TP_4545 = smd 1.143 x 1.143: T 0,0
HE50 = smd 1.2 x 2.3: 1 -19.05,12.55; 2 -16.51,12.55; 3 -13.97,12.55; 4 -11.43,12.55; 5 -8.89,12.55; 6 -6.35,12.55; 7 -3.81,12.55; 8 -1.27,12.55; 9 1.27,12.55; 10 3.81,12.55; 11 6.35,12.55; 12 8.89,12.55; 13 11.43,12.55; 14 13.97,12.55; 15 16.51,12.55; 16 19.05,12.55; 26 19.05,-12.55; 27 16.51,-12.55; 28 13.97,-12.55; 29 11.43,-12.55; 30 8.89,-12.55; 31 6.35,-12.55; 32 3.81,-12.55; 33 1.27,-12.55; 34 -1.27,-12.55; 35 -3.81,-12.55; 36 -6.35,-12.55; 37 -8.89,-12.55; 38 -11.43,-12.55; 39 -13.97,-12.55; 40 -16.51,-12.55; 41 -19.05,-12.55 | smd 2.3 x 1.2: 17 21.45,10.05; 18 21.45,7.51; 19 21.45,4.97; 20 21.45,2.43; 21 21.45,-0.11; 22 21.45,-2.65; 23 21.45,-5.19; 24 21.45,-7.73; 25 21.45,-10.27; 42 -21.45,-10.27; 43 -21.45,-7.73; 44 -21.45,-5.19; 45 -21.45,-2.65; 46 -21.45,-0.11; 47 -21.45,2.43; 48 -21.45,4.97; 49 -21.45,7.51; 50 -21.45,10.05
PDSO-G8 = smd 0.25 x 0.9: 1 -0.975,-1.9; 2 -0.325,-1.9; 3 0.325,-1.9; 4 0.975,-1.9; 5 0.975,1.9; 6 0.325,1.9; 7 -0.325,1.9; 8 -0.975,1.9
SOT23-5 = smd 0.69 x 1.2: 1 -0.95,-1.3; 2 0,-1.3; 3 0.95,-1.3; 4 0.95,1.3; 5 -0.95,1.3
QFN44 = smd 1 x 0.3: 1 -3.35,2.5; 2 -3.35,2; 3 -3.35,1.5; 4 -3.35,1; 5 -3.35,0.5; 6 -3.35,0; 7 -3.35,-0.5; 8 -3.35,-1; 9 -3.35,-1.5; 10 -3.35,-2; 11 -3.35,-2.5; 23 3.35,-2.5; 24 3.35,-2; 25 3.35,-1.5; 26 3.35,-1; 27 3.35,-0.5; 28 3.35,0; 29 3.35,0.5; 30 3.35,1; 31 3.35,1.5; 32 3.35,2; 33 3.35,2.5 | smd 0.3 x 1: 12 -2.5,-3.35; 13 -2,-3.35; 14 -1.5,-3.35; 15 -1,-3.35; 16 -0.5,-3.35; 17 0,-3.35; 18 0.5,-3.35; 19 1,-3.35; 20 1.5,-3.35; 21 2,-3.35; 22 2.5,-3.35; 34 2.5,3.35; 35 2,3.35; 36 1.5,3.35; 37 1,3.35; 38 0.5,3.35; 39 0,3.35; 40 -0.5,3.35; 41 -1,3.35; 42 -1.5,3.35; 43 -2,3.35; 44 -2.5,3.35 | smd 5.08 x 5.08: TAB 0,0
2P-SMD-5X3.2 = smd 1.778 x 2.032: 1 -2.159,0; 2 2.159,0

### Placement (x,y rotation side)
C1  20.95,44.45 0 top
C2  20.95,38.1 0 top
C3  31.37,24.89 180 bottom
C4  24.13,38.1 0 top
C5  60.26,39.37 180 bottom
C6  58.55,29.97 270 bottom
C7  52.2,30.73 90 bottom
C8  45.09,10.79 270 bottom
C9  57.79,16.51 270 bottom
C10  16.89,13.72 180 bottom
C11  58.67,22.23 270 bottom
C12  52.2,22.99 90 bottom
C13  32.99,14.48 90 bottom
C14  39.65,14.48 90 bottom
C15  35.18,24.89 0 bottom
C16  42.42,21.97 0 bottom
C17  35.31,14.48 90 bottom
C18  30.23,19.81 180 bottom
C19  40.51,27.43 270 bottom
C20  32.89,27.43 270 bottom
C21  12.45,29.84 270 top
C22  11.3,29.84 270 top
C23  58.67,26.16 270 bottom
C24  52.2,26.92 90 bottom
C25  50.29,14.35 90 bottom
C26  55.88,16.51 270 bottom
C27  53.34,17.14 90 bottom
D1  38.73,5.71 180 bottom
D3  16.51,9.53 90 bottom
D6  8.76,26.99 90 bottom
F2  8.26,29.84 0 top
I2C  46.99,39.37 270 top
ICSP  64.77,27.94 0 top
J1  1.78,41.27 270 top
J2  12.7,9.53 180 top
J3  54.61,50.8 270 top
J4  30.23,50.8 270 top
J5  57.15,2.54 90 top
J7  36.83,2.54 270 top
J8  4.45,24.77 270 top
L  8.26,24.51 0 top
L3  53.34,11.43 90 bottom
LAN  66.67,22.86 0 top
MISO  34.93,45.72 0 bottom
MOSI  40.01,45.72 0 bottom
ORST  66.55,13.97 90 top
P1  66.04,4.45 0 top
P2  63.63,5.08 0 bottom
P3  3.81,51.44 0 bottom
P4  5.08,51.44 0 top
PWR  25.02,1.91 270 top
Q1  47.62,17.78 270 bottom
Q2  25.65,21.59 270 bottom
R1  11.43,19.56 0 bottom
R2  20.95,41.66 180 top
R3  63.5,17.91 180 bottom
R4  26.92,23.88 0 bottom
R5  20.95,43.43 180 top
R6  28.19,21.97 270 bottom
R8  24.13,39.12 180 top
R9  24.13,40.89 180 top
R10  60.26,38.1 0 bottom
R11  25.02,4.45 270 bottom
R12  63.5,22.86 180 bottom
R13  63.56,21.21 180 bottom
R14  63.5,19.56 180 bottom
R15  52.2,28.83 90 bottom
R16  48.77,14.35 90 bottom
R17  47.24,14.35 90 bottom
R18  50.42,18.67 180 bottom
R19  50.42,16.89 180 bottom
R20  52.2,21.08 90 bottom
R22  14.35,4.45 270 bottom
R23  33.27,24.89 0 bottom
R24  11.43,24.51 180 bottom
R25  11.43,22.86 0 bottom
R26  11.43,27.81 180 bottom
R27  11.43,26.16 180 bottom
R28  11.43,21.21 0 bottom
R29  52.2,25.02 90 bottom
RESET  19.68,2.03 0 top
RST  14.35,1.91 270 top
RX  8.26,22.86 0 top
SCK  29.84,45.72 0 bottom
SCL  34.93,10.16 270 bottom
SDA  37.47,10.16 270 bottom
START  64.01,43.18 90 top
SYS  66.67,19.56 0 top
TP1  22.86,6.99 0 bottom
TP2  22.86,4.45 0 bottom
TP3  22.86,1.91 0 bottom
TX  8.26,21.21 0 top
U2  38.73,19.68 0 top
U3  55.37,29.84 270 bottom
U4  48.64,10.79 270 bottom
U5  55.5,22.1 270 bottom
U7  36.83,19.68 180 bottom
U8  55.5,26.04 270 bottom
U$1  [OSHW_FILLX200_NOTEXT]  29.21,37.47 0 bottom
U$2  [LOGO_SILK]  18.41,39.37 0 bottom
UART  55.88,39.37 270 top
USB  8.26,19.56 0 top
WLAN  66.67,21.21 0 top
X1  36.68,27.38 180 bottom

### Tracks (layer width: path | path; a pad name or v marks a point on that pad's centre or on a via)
3V3  (via drill 0.3 pad 0.64)
  Top 0.406: U2.23 60.2,14.48 60.33,14.48 62.1,14.48 63.06,15.43 v63.06,17.14 v63.06,22.04
  Top 0.813: U2.24 58.28,11.96 57.79,12.45 v57.79,14.35 60.2,14.35 60.33,14.48 | J7.5 35.69,2.54 36.2,3.05 36.2,9.02 36.83,9.65 39.88,9.65 v50.93,20.7
  Bottom 0.203: U8.3 C23.2 | U3.3 C6.2 | C11.2 U5.3 | R3.1 v63.06,17.14 | v63.06,22.04 R12.1
  Bottom 0.305: R11.1 33.21,4.89 J7.5
  Bottom 0.61: C6.2 59.27,29.53 | 59.27,29.53 59.37,29.53 59.82,29.08 | 59.82,29.08 59.82,25.65 | 59.82,25.65 59.82,25.27 | 59.82,25.27 59.82,22.1 | 59.82,22.1 59.82,21.84 | 59.82,21.84 59.82,21.46 | 59.82,21.46 59.82,20.19 | 59.82,20.19 59.82,19.94 | 59.82,19.94 59.82,19.43 | 59.82,19.43 59.82,16.26 59.18,15.62 C9.2 | C23.2 59.27,25.72 | 59.27,25.72 59.75,25.72 59.82,25.65 | C11.2 59.39,21.78 | 59.39,21.78 59.75,21.78 59.82,21.84 | v50.93,20.7 51.82,19.81 59.33,19.81 | 59.33,19.81 59.69,19.81 59.82,19.94 | 59.82,29.08 59.82,29.97 | 59.82,29.97 R10.2 | 59.27,29.53 arc45 59.45,29.6 59.82,29.97 | 59.27,25.72 arc45 59.45,25.79 59.69,26.04 | 59.27,25.72 arc-45 59.45,25.64 59.82,25.27 | 59.39,21.78 arc45 59.57,21.86 59.82,22.1 | 59.39,21.78 arc-45 59.57,21.71 59.82,21.46 | 59.33,19.81 arc45 59.51,19.89 59.82,20.19 | 59.33,19.81 arc-45 59.51,19.74 59.82,19.43
  Bottom 0.813: v57.79,14.35 C9.2 C26.2 53.4,15.62 C27.+ | R16.2 C25.2 50.8,15.11 51.31,15.62 53.28,15.62 C27.+ | L3.2 C27.+
5V  (via drill 0.3 pad 0.64, 0.3 pad 0.81)
  Top 0.406: TX.+ v7.49,22.04 RX.+
  Top 0.61: ICSP.6 66.04,31.11 60.71,36.45 57.8,36.45 | 57.8,36.45 57.79,36.45 | 32.02,15.61 v32,15.62 | 57.8,36.45 UART.3 | v34.16,24.89 32,22.73 v32,20.19 v32,17.53 | v41.91,22.73 41.91,17.4 v40.7,16.19
  Top 0.813: J7.4 41.27,5.71 41.27,8.43 42.76,9.91 v43.82,9.91 | I2C.3 UART.3 | 32.02,15.61 40.12,15.61 v40.7,16.19 | 14.35,16.26 v14.35,22.04 14.35,29.21 13.27,30.29 C21.1 C22.1 10.1,30.29 F2.2 | 14.35,16.26 14.35,15.75 | v32,15.62 v32,17.53 | v19.05,15.75 14.86,15.75 | 14.86,15.75 14.35,15.75 | 14.35,15.24 v14.35,13.03 v14.35,6.35 | 14.86,15.75 14.35,16.26 | 14.86,15.75 14.35,15.24 | 14.35,15.24 14.35,15.75
  Bottom 0.203: U7.34 39.33,15.24 C14.2 | U7.7 v32.01,20.18 v32,20.19 | U7.2 32.16,17.68 v32,17.53 | v41.91,22.73 41.97,22.67 C16.2 41.69,21.68 U7.24 | U3.7 52.32,30.17 C7.1 | C15.2 34.73,24.45 35.33,23.85 U7.14 | U5.7 52.32,22.42 C12.1 | U8.7 52.32,26.36 C24.1 | U4.1 48.7,11.74 48.26,11.3 48.26,10.03 48.07,9.85 U4.4
  Bottom 0.305: U7.44 34.33,16.13 34.29,16.13 33.15,14.99 33.06,14.99 C13.2
  Bottom 0.406: v14.35,22.04 v7.49,22.04 | v14.35,6.35 R22.1
  Bottom 0.61: R23.1 v34.16,24.89 C15.2 | C12.1 49.34,22.54 | 49.34,22.54 48.64,21.84 | 48.64,21.84 43.05,16.26 40.77,16.26 v40.7,16.19 | 48.64,21.84 48.64,22.99 | 48.64,22.99 48.64,26.16 | 48.64,26.16 48.64,26.8 | 48.64,26.8 48.64,29.97 | 48.64,29.97 48.64,30.61 | 48.64,30.61 48.64,31.52 arc-45 48.72,31.7 55.37,38.35 55.84,38.35 arc45 UART.3 | 49.34,22.54 49.09,22.54 48.64,22.99 | C24.1 48.96,26.48 | 48.96,26.48 48.64,26.8 | 48.96,26.48 48.64,26.16 | C7.1 48.96,30.29 | 48.96,30.29 48.64,30.61 | 48.96,30.29 48.64,29.97 | C14.2 40.26,14.92 | 40.26,14.92 40.7,15.37 | 40.26,14.92 40.32,14.92 40.77,14.48 | C13.2 32.7,14.92 v32,15.62 31.88,15.75 v19.05,15.75
  Bottom 0.813: U4.4 45.15,9.85 C8.2 v43.82,9.91 40.7,13.02 40.7,15.37 v40.7,16.19 | J7.7 32,1.02 36.58,1.02 J7.4 38.1,4.7 D1.+ | C10.+ 15.49,13.65 15.49,13.21 15.37,13.08 15.31,13.03 v14.35,13.03 J2.+
5V_OUT
  Bottom 0.61: J7.1 45.34,2.54 43.94,3.94 42.16,3.94 D1.-
!RESET  (via drill 0.3 pad 0.64)
  Top 0.203: J7.6 33.66,3.17 33.66,4.95 | 33.66,4.95 33.66,5.08 | 33.66,5.08 33.66,5.21 | 33.66,5.21 33.66,8.76 | 33.66,8.76 33.66,8.89 | v32.39,24.89 31.24,23.75 31.24,14.86 v31.37,14.73 | v32.26,8.89 33.53,8.89 | 33.53,8.89 33.66,8.89 | 33.66,8.89 33.78,8.89 | 33.78,8.89 34.93,8.89 36.58,10.54 39.64,10.54 48.77,19.67 v48.77,20.07 49.28,20.07 50.6,21.39 58.24,21.39 58.8,20.83 61.34,20.83 61.72,21.21 61.72,23.62 ICSP.3 | 33.66,8.76 33.53,8.89 | 33.66,8.76 33.78,8.89 | RST.- 13.34,2.16 13.34,4.45 13.97,5.08 21.72,5.08 | 21.72,5.08 21.84,5.08 | 21.97,5.08 33.27,5.08 33.53,5.08 | 33.53,5.08 33.66,5.08 | RESET.2 21.84,4.95 | 21.84,4.95 21.84,5.08 | 21.97,5.08 21.84,4.95 | 21.84,4.95 21.72,5.08 | 21.84,5.08 21.97,5.08 | 33.53,5.08 33.66,5.21 | 33.53,5.08 33.66,4.95
  Bottom 0.203: U7.13 34.83,23.72 34.42,24.13 33.02,24.13 32.83,24.32 R23.2 | Q1.3 46.74,17.78 46.74,18.87 47.93,20.07 v48.77,20.07 | v32.26,8.89 31.37,9.78 v31.37,14.73
  Bottom 0.406: C3.2 v32.39,24.89 R23.2
AREF  (via drill 0.3 pad 0.64)
  Top 0.406: v30.48,21.59 30.48,14.61 31.11,13.97 33.97,13.97 v34.67,14.67
  Bottom 0.203: U7.42 35.33,14.95 C17.2 35.05,14.67 v34.67,14.67
  Bottom 0.406: J4.8 27.07,47.6 27.07,36.85 25.02,34.8 25.02,25.38 25.76,24.64 27.81,24.64 30.48,21.97 v30.48,21.59
CTRL_2.0V
  Top 0.406: U2.2 22.22,34.92 20.51,36.64 C2.1 J1.P1 14.48,38.1 14.1,38.48 14.1,44.07 14.48,44.45 J1.P6
D14/PB3/MISO  (via drill 0.3 pad 0.64)
  Top 0.203: ICSP.1 63.5,32.15 60.73,34.92 41.15,34.92 35.37,40.7 v35.37,41.21 | v60.96,23.5 v58.42,23.5
  Bottom 0.203: U7.11 32.04,22.18 26.67,27.56 26.67,33.91 33.72,40.96 35.12,40.96 v35.37,41.21 36.2,42.04 MISO.00 | ICSP.1 60.96,27.94 v60.96,23.5 | U5.1 58,23.07 v58.42,23.5
D15/PB1/SCK  (via drill 0.3 pad 0.64)
  Top 0.203: ICSP.2 62.1,29.34 62.1,32.86 60.42,34.54 54.23,34.54 | v31.11,41.4 34.16,41.4 41.02,34.54 53.72,34.54 | 53.98,34.54 54.23,34.54 | 53.98,34.29 53.98,29.72 52.32,28.07 52.32,24.77 v52.96,24.13 | 53.98,34.29 53.98,34.54 | 53.72,34.54 53.98,34.29 | 53.98,34.29 54.23,34.54 | 53.98,34.54 53.72,34.54
  Bottom 0.203: U7.9 32.66,21.18 32.51,21.34 31.88,21.34 25.91,27.3 25.91,34.29 31.11,39.5 v31.11,41.4 SCK.00 | U5.8 53.6,23.49 v52.96,24.13
D16/PB2/MOSI  (via drill 0.3 pad 0.64)
  Top 0.203: v40.01,43.05 v35.31,43.05 | v41.02,36.07 41.78,35.31 60.93,35.31 64.77,31.46 64.77,29.21 ICSP.5 64.77,26.67 62.99,26.67 61.09,28.57 58.17,28.57 56.9,27.3 v54.61,27.3
  Bottom 0.203: U7.10 32.8,21.68 32.77,21.72 32,21.72 26.29,27.43 26.29,34.04 v35.31,43.05 | MOSI.00 41.27,44.32 v40.01,43.05 40.01,40.39 41.4,38.99 41.4,36.45 v41.02,36.07 | U8.8 54.32,27.01 v54.61,27.3
D17/PB0/RXLED/SS  (via drill 0.3 pad 0.64)
  Top 0.203: v29.21,21.59 29.84,20.95 29.84,14.35 32.51,11.68 39.24,11.68 46.36,18.8 46.36,22.23 46.99,22.86 55.88,22.86 56.77,23.75 v56.9,23.75
  Bottom 0.203: U7.8 32.53,20.68 32.26,20.95 29.84,20.95 v29.21,21.59 29.21,22.1 28.89,22.42 R6.1 28.19,23.5 27.81,23.88 R4.1 | U8.1 56.86,27.01 56.64,26.8 56.64,24 v56.9,23.75
D+
  Bottom 0.203: U7.4 25.13,18.68 23.62,20.19 23.62,25.21 21.65,27.18 12.51,27.18 R26.2
D-
  Bottom 0.203: R27.2 12.51,26.8 21.46,26.8 23.24,25.02 23.24,20 25.06,18.18 U7.3
GND  (via drill 0.3 pad 0.64)
  Top 0.203: U2.42 17.42,9.41 D3.3
  Bottom 0.203: U7.35 38.83,14.38 39.18,14.03 C14.1 | C18.1 30.23,19.05 32.77,19.05 32.9,19.18 U7.5 34.43,19.18 v34.93,19.68 | v34.93,17.78 34.83,17.68 U7.43 34.83,15.78 34.04,14.99 34.04,13.59 v34.29,13.34 | v34.93,21.59 35.43,21.59 35.83,21.99 U7.15 35.83,24.75 35.69,24.89 | U7.23 39.33,22.18 v38.73,21.59 | U7.33 39.33,17.18 v38.73,17.78 | U5.2 v58.11,22.42 | C11.1 58.43,22.42 v58.11,22.42 | U8.2 58.43,26.36 C23.1 | v58.11,22.42 v58.1,22.42
  Bottom 0.305: R20.1 52.01,20.64 51.31,21.34
  other vias: 39.12,14.22 10.16,32.38 19.05,25.4 29.21,17.59 27.81,30.42 27.81,28.89 29.21,28.89 30.48,28.89 31.75,28.89 33.02,28.89 33.02,30.42 34.8,30.42 34.93,28.89 36.2,28.89 37.47,28.89 38.73,28.89 40.01,28.89 41.15,28.89 41.15,30.54 41.15,31.81 41.15,33.08 40.01,34.29 38.73,34.29 37.47,34.29 36.2,35.56 36.2,38.1 33.66,38.1 31.88,40.64 29.84,42.29 26.04,43.81 24.76,43.81 23.49,43.81 22.22,43.81 22.22,41.78 23.49,41.78 24.76,41.78 26.04,41.78 27.94,41.27 27.94,43.88 29.53,39.62 31.75,37.47 32.96,36.13 34.23,34.73 33.66,32.45 32.39,34.73 31.11,34.73 29.84,34.73 25.53,39.18 26.04,38.54 27.81,33.59 18.41,43.81 18.41,41.78 18.41,40.89 18.41,39.12 19.94,39.24 21.97,39.24 36.83,19.68 36.83,21.59 38.73,19.68 36.83,17.78 40.26,22.99 41.27,23.5 42.55,23.5 33.02,12.7 42.93,22.73 31.75,27.3 30.48,27.3 29.21,27.3 35.69,24.38 46.36,8.89 45.72,12.7 49.02,10.79 47.62,8.89 49.4,12.7 48.9,16.13 50.8,17.78 53.34,17.78 52.07,17.78 54.61,17.78 55.88,18.41 57.15,18.41 58.42,18.41 55.88,13.97 55.88,12.7 55.88,11.43 55.88,10.16 57.15,11.43 57.15,10.16 60.96,15.88 67.44,20.38 58.93,31.11 22.22,19.68 22.22,17.14 22.86,14.61 22.86,12.83 25.4,14.61 27.94,14.61 27.94,12.7 25.4,12.7 19.05,18.41 27.94,8.89 19.05,20.32 19.68,3.81 22.86,10.79 22.86,8.89 25.4,10.79 25.4,8.89 34.93,4.45 23.49,27.94 15.88,6.99 16.51,3.81 17.78,6.99 58.42,10.16 15.24,30.48 17.78,33.66 17.78,36.2 19.68,36.2 19.68,33.66 23.49,33.66 23.49,36.2 22.22,36.2 22.22,37.47 24.76,36.2 26.04,37.47 24.76,45.72 26.04,45.72 23.49,45.72 22.22,45.72 20.95,45.72 18.41,45.72 19.68,45.72 18.41,47.62 20.95,47.62 23.49,47.62 50.16,29.21 50.16,27.43 50.16,25.4 50.16,23.5 12.45,28.7 11.3,28.7 37.47,40.01 38.73,40.64 38.73,38.73 40.01,39.37 40.01,37.47 58.42,43.81 59.69,43.81 58.42,45.09 23.49,34.92 17.78,34.92 59.69,45.09 55.88,29.84 54.61,29.84 58.42,27.94 15.24,32.38 37.47,36.83 38.73,35.56 34.93,36.83 34.93,39.37 66.17,17.91 63.75,11.81 64.52,13.97 26.04,1.27 10.16,24.51 10.16,19.56 8.89,26.99 10.79,26.99 15.49,25.4 12.7,25.4 12.7,20.32 19.05,9.53 32.39,43.81 3.17,19.68 3.17,29.84 15.49,17.02 19.68,14.61 24.76,24.13
  pour Top (isolate 0.254, rank 6): -0.64,53.98 69.21,53.98 69.21,0 -0.64,0
  pour Bottom (isolate 0.254, rank 6): -0.64,53.98 69.21,53.98 69.21,0 -0.64,0
  pour Top (isolate 0.254, no thermals): -0.64,53.98 8.26,53.98 8.26,0 -0.64,0
GPIO18  (via drill 0.3 pad 0.64)
  Top 0.203: U2.18 58.56,27.2 57.28,25.91 v54.86,25.91
  Bottom 0.203: U5.5 54.65,21.12 55.12,21.59 55.12,25.65 v54.86,25.91
GPIO19  (via drill 0.3 pad 0.64)
  Top 0.203: U2.19 59.91,24.38 57.91,24.38 56.9,25.4 55.18,25.4 v54.55,24.77
  Bottom 0.203: R29.2 52.44,25.71 U8.6 54.2,25.71 54.74,25.17 54.74,24.77 | R20.2 52.44,21.77 U5.6 54.36,21.77 54.74,22.15 54.74,24.77 | v54.55,24.77 54.74,24.77
GPIO20  (via drill 0.3 pad 0.64)
  Top 0.203: U2.20 58.69,22.11 58.42,21.84 50.16,21.84 v49.4,21.08
  Bottom 0.203: v49.4,21.08 49.4,20.19 50.67,18.92 50.67,18.86 R18.2
GPIO21  (via drill 0.3 pad 0.64)
  Top 0.203: v52.96,25.02 52.96,26.57 54.33,27.94 55.75,27.94 57.79,29.97 U2.16
  Bottom 0.203: U8.5 53,25.06 v52.96,25.02
GPIO22  (via drill 0.3 pad 0.64)
  Top 0.203: U2.17 58.44,29.73 v56.64,27.94
  Bottom 0.203: U5.4 56.73,21.12 56.26,21.59 56.26,27.56 v56.64,27.94
GPIO23  (via drill 0.3 pad 0.64)
  Top 0.203: v58.17,25.02 59.18,26.04 v61.59,26.04 | v60.96,18.41 60.96,19.43 60.83,19.56 60.2,19.56 U2.21
  Bottom 0.203: U8.4 58.12,25.06 v58.17,25.02 | v61.59,26.04 61.59,22.86 60.96,22.23 v60.96,18.41
GPIO24  (via drill 0.3 pad 0.64)
  Top 0.203: U2.3 24.76,29.97 26.51,28.23 51.54,28.23 v52.83,29.52
  Bottom 0.203: U3.6 v52.83,29.52 52.44,29.52 R15.2
GPIO28  (via drill 0.3 pad 0.64)
  Top 0.203: v56.52,7.62 55.25,7.62 55.12,7.62
  Top 0.406: U2.27 55.25,7.62
  Bottom 0.203: 63.06,19.49 R14.1 62.23,18.73 62.23,9.14 60.71,7.62 v56.52,7.62
JUMPSTART  (via drill 0.3 pad 0.64)
  Top 0.203: U2.37 29.84,9.14 31.62,10.92 39.5,10.92 47.75,19.18 v47.75,22.23 | v57.15,39.37 58.8,41.02 v60.71,41.02 61.21,41.02 START.1 62.1,40.64
  Bottom 0.203: v47.75,22.23 47.75,31.62 55.5,39.37 v57.15,39.37 | R10.1 C5.2 v60.71,41.02
LED0_WLAN  (via drill 0.3 pad 0.64)
  Top 0.203: U2.30 47.62,7.62 48.26,8.26 v48.9,8.26
  Bottom 0.203: v48.9,8.26 60.45,8.26 61.59,9.4 61.59,19.68 R13.1
LED1_USB  (via drill 0.3 pad 0.64)
  Top 0.203: U2.29 50.16,5.74 50.02,5.59 43.18,5.59 v42.93,5.33
  Bottom 0.203: v42.93,5.33 42.93,5.97 41.66,7.24 32,7.24 27.18,12.06 17.78,12.06 16.51,13.34 16.51,17.91 14.86,19.56 R1.1
LED2_P0  (via drill 0.3 pad 0.64)
  Top 0.203: v67.44,23.62 LAN.- | v46.36,6.99 45.23,6.99 U2.31
  Bottom 0.203: v46.36,6.99 60.96,6.99 65.41,11.43 65.41,21.59 v67.44,23.62
N$1
  Bottom 0.203: C19.2 39.23,26.99 38.95,27.27 | 38.95,27.27 X1.2 | U7.17 36.83,25.15 38.95,27.27
N$2
  Bottom 0.203: C20.2 34.12,26.99 X1.1 35.05,26.85 35.05,26.8 36.33,25.52 U7.16
N$4  (via drill 0.3 pad 0.64)
  Top 0.203: v10.98,23.75 8.26,23.75 L.+
  Bottom 0.203: R24.1 v10.98,23.75
N$5  (via drill 0.3 pad 0.64)
  Top 0.203: v10.16,21.21 TX.-
  Bottom 0.203: R28.2 v10.16,21.21
N$6  (via drill 0.3 pad 0.64)
  Top 0.203: J8.2 5.1,25.41 5.33,25.65 5.71,25.65 5.97,25.4 v6.35,25.4
  Bottom 0.203: R27.1 7.81,26.16 D6.1 | D6.1 7.68,26.1 | v6.35,25.4 6.35,25.53 6.1,25.78 6.1,26.54 6.36,26.81 7.04,26.81 D6.1
N$7  (via drill 0.3 pad 0.64)
  Top 0.203: v22.61,22.86 v25.4,22.86
  Bottom 0.203: R6.2 27.5,21.53 Q2.2 26.54,20.7 26.54,20.83 25.65,21.72 25.65,22.61 v25.4,22.86 | v22.61,22.86 R25.1
N$8  (via drill 0.3 pad 0.64)
  Top 0.203: J8.3 5.27,24.77 v5.53,25.02
  Bottom 0.203: R26.1 7.81,27.81 D6.2 7.68,27.88 6.99,27.18 6.22,27.18 5.71,26.67 5.71,25.21 v5.53,25.02
N$9
  Bottom 0.406: 50.16,9.78 50.01,9.78 U4.3
  Bottom 0.813: L3.1 50.55,9.4 50.16,9.78
  pour Bottom (isolate 0.254, no thermals): 49.4,10.1 54.61,10.1 arc-90 54.86,9.84 54.86,8.95 arc-90 54.61,8.7 50.33,8.7 arc-45 50.15,8.77 49.48,9.45 arc-45 49.4,9.63
N$10  (via drill 0.3 pad 0.64)
  Top 0.203: v10.98,20.38 8.32,20.38 USB.+
  Bottom 0.203: R1.2 v10.98,20.38
N$11
  Bottom 0.406: C25.1 R16.1 R17.1 47.24,11.84 U4.5
N$12
  Top 0.203: 4.6,26.07 4.73,26.07
  Top 0.305: J8.1 4.6,26.07 | 4.73,26.07 4.73,26.29 4.73,26.39
  Top 0.813: F2.1 5.59,28.57 5.59,26.8 5.08,26.29 4.73,26.29 4.7,26.29
N$13
  Bottom 0.203: Q1.1 R18.1 R19.1
N$14  (via drill 0.3 pad 0.64)
  Top 0.203: R2.2 v19.94,41.66 | v19.94,43.43 R5.2 C1.1
  Bottom 0.203: v19.94,41.66 v19.94,43.43
N$15  (via drill 0.3 pad 0.64)
  Top 0.203: 17.3,11.94 U2.43 15.83,11.96 v15.81,11.94 | v43.69,4.83 44.07,5.21 61.09,5.21 62.87,6.99 62.87,14.1 64.77,16 | 64.77,16 64.9,16 ORST.2 | v64.77,17.91 64.77,16
  Bottom 0.203: v43.69,4.83 43.56,4.7 42.69,4.7 42.29,5.1 42.29,5.97 41.4,6.86 31.88,6.86 27.05,11.68 16.07,11.68 v15.81,11.94 | v64.77,17.91 R3.2
N$16  (via drill 0.3 pad 0.64)
  Top 0.203: v10.16,22.86 RX.-
  Bottom 0.203: R25.2 v10.16,22.86
N$17  (via drill 0.3 pad 0.64)
  Top 0.203: v14.35,3.37 RST.+
  Bottom 0.203: R22.2 v14.35,3.37
N$18  (via drill 0.3 pad 0.64)
  Top 0.203: C4.1 R8.2 v22.86,39.12 | R9.2 v22.86,40.89
  Bottom 0.203: v22.86,40.89 v22.86,39.12
N$19
  Bottom 0.203: R4.2 26.48,22.67 Q2.1
N$23  (via drill 0.3 pad 0.64)
  Top 0.203: v25.02,3.37 PWR.+
  Bottom 0.203: R11.2 v25.02,3.37
N$24  (via drill 0.3 pad 0.64)
  Top 0.203: LAN.+ v64.77,22.86
  Bottom 0.203: v64.77,22.86 R12.2
N$25  (via drill 0.3 pad 0.64)
  Top 0.203: v64.01,22.04 65.09,22.04 WLAN.+
  Bottom 0.203: v64.01,22.04 R13.2
N$26  (via drill 0.3 pad 0.64)
  Top 0.203: 66.04,19.43 SYS.+ v64.77,19.56
  Bottom 0.203: v64.77,19.56 R14.2
P0_RX+
  Top 0.152: J1.P4 17.4,41.91 17.88,42.39 21.24,42.39 | 21.56,42.39 27.83,42.39 36.04,34.18 36.04,30.07 36.58,29.53 38.35,29.53 38.93,30.1 38.93,30.61 40.01,31.69 U2.9 | 21.56,42.39 21.4,42.39 | 21.4,42.39 21.24,42.39 | R2.1 21.4,42.23 | 21.4,42.23 21.4,42.39 | 21.24,42.39 21.4,42.23 | 21.56,42.39 21.4,42.23
P0_RX-
  Top 0.152: J1.P5 17.4,43.18 17.88,42.7 21.24,42.7 | 21.24,42.7 21.4,42.7 | 21.4,42.7 21.56,42.7 | 21.56,42.7 27.98,42.7 36.35,34.33 36.35,30.2 36.7,29.84 37.01,29.84 arc90 37.21,30.05 37.21,30.09 arc-90 37.41,30.29 37.52,30.29 arc-90 37.72,30.09 37.72,30.05 arc90 37.92,29.84 38.23,29.84 38.54,30.16 38.54,30.61 37.47,31.69 U2.8 | R5.1 21.4,42.86 | 21.4,42.86 21.4,42.7 | 21.24,42.7 21.4,42.86 | 21.56,42.7 21.4,42.86
P0_TX+
  Top 0.152: J1.P2 17.4,39.37 17.88,39.85 24.42,39.85 | 24.42,39.85 24.57,39.85 | 24.57,39.85 24.73,39.85 | 24.73,39.85 25.94,39.85 28.42,37.37 28.42,30.07 28.96,29.53 30.73,29.53 31.31,30.1 31.31,30.61 32.39,31.69 U2.6 | R8.1 24.57,39.69 | 24.57,39.69 24.57,39.85 | 24.42,39.85 24.57,39.69 | 24.73,39.85 24.57,39.69
P0_TX-
  Top 0.152: J1.P3 17.4,40.64 17.88,40.16 24.42,40.16 | 24.42,40.16 24.57,40.16 | 24.57,40.16 24.73,40.16 | 24.73,40.16 26.07,40.16 28.73,37.5 28.73,30.19 29.08,29.84 29.4,29.84 arc90 29.59,30.04 29.59,30.1 arc-90 29.78,30.29 29.91,30.29 arc-90 30.1,30.1 30.1,30.04 arc90 30.29,29.84 30.61,29.84 30.92,30.16 30.92,30.61 29.84,31.69 U2.5 | R9.1 24.57,40.32 | 24.57,40.32 24.57,40.16 | 24.73,40.16 24.57,40.32 | 24.42,40.16 24.42,40.17 24.57,40.32
PB4/A8/D8  (via drill 0.3 pad 0.64)
  Top 0.203: v49.53,47.62 44.83,47.62 J4.1
  Bottom 0.203: U7.28 43.16,19.68 44.96,21.48 44.96,32.38 48.64,36.07 48.64,46.74 v49.53,47.62
PB5/A9/D9  (via drill 0.3 pad 0.64)
  Top 0.203: v49.53,46.74 43.18,46.74 J4.2
  Bottom 0.203: U7.29 43.19,19.18 45.34,21.34 45.34,32.13 49.02,35.81 49.02,46.23 v49.53,46.74
PB6/A10/D10  (via drill 0.3 pad 0.64)
  Top 0.203: v49.66,45.85 41.53,45.85 J4.3
  Bottom 0.203: U7.30 43.3,18.68 45.72,21.1 45.72,32 49.4,35.69 49.4,45.59 v49.66,45.85
PB7/D11
  Bottom 0.203: U7.12 34.33,23.58 34.16,23.75 30.99,23.75 27.05,27.69 27.05,33.66 33.91,40.51 35.55,40.51 38.73,43.7 MOSI.11 MOSI.MM 40.01,46.74 39.62,47.12 37.72,47.12 J4.4
PC7/D13  (via drill 0.3 pad 0.64)
  Top 0.203: v26.04,25.4 23.49,25.4 v22.61,24.51 | v50.8,45.21 30.99,45.21 v28.57,47.62
  Bottom 0.203: U7.32 43.43,17.68 46.48,20.74 46.48,31.62 50.16,35.31 50.16,44.58 v50.8,45.21 | SCK.11 28.57,37.59 25.53,34.54 25.53,25.91 v26.04,25.4 | SCK.11 SCK.MM 29.84,49.91 J4.6 | R24.2 v22.61,24.51 | SCK.11 v28.57,47.62
PD0/SCL/D3  (via drill 0.3 pad 0.64)
  Top 0.203: v41.4,26.04 42.19,26.04 44.83,23.39 44.83,17.78 39.12,12.06 34.29,12.06 v33.91,12.45 | v52.2,42.42 52.15,42.37 I2C.1 40.89,42.37 v40.64,42.37 31.54,42.37 25.02,48.9 20.7,48.9 J4.10
  Bottom 0.203: U7.18 37.33,24.26 38.59,25.53 40.89,25.53 v41.4,26.04 41.78,26.42 41.78,39.24 40.64,40.39 v40.64,42.37 | v52.2,42.42 52.2,43.43 55.88,47.12 J3.4 | 34.04,8.89 33.66,9.27 33.66,12.19 v33.91,12.45
  Bottom 0.406: SCL.11 34.04,8.89
PD1/SDA/D2  (via drill 0.3 pad 0.64)
  Top 0.203: v41.91,25.4 44.32,22.99 44.32,17.78 39.24,12.7 v36.2,12.7 | v52.83,40.39 47.01,40.39 I2C.2 42.02,40.37 v41.91,40.26 40.26,41.91 31.5,41.91 24.89,48.51 19.18,48.51 17.54,50.15 17.54,51.32 18.16,51.94 20.19,51.94 J4.9
  Bottom 0.203: U7.19 37.83,24.14 38.83,25.15 41.66,25.15 v41.91,25.4 42.16,25.65 42.16,40.01 v41.91,40.26 | J3.3 58.42,49.02 52.83,43.43 v52.83,40.39 | v36.2,12.7 36.45,12.45 36.45,9.14 36.7,8.89
  Bottom 0.406: 36.7,8.89 SDA.11
PD2/RXI/D0  (via drill 0.3 pad 0.64)
  Top 0.203: v43.18,41.27 54.79,41.27 UART.1
  Bottom 0.203: U7.20 38.33,24.03 39.07,24.77 42.29,24.77 42.55,25.02 42.55,40.64 v43.18,41.27 | J3.1 62.23,49.53 60.45,49.53 55.88,44.96 UART.1 57.79,40.47 57.79,34.29 54.32,30.82 U3.8
PD3/TXO/D1  (via drill 0.3 pad 0.64)
  Top 0.203: v43.18,39.37 54.88,39.37 UART.2 57.42,41.91 v57.79,41.91
  Bottom 0.203: U7.21 38.83,23.82 39.39,24.38 42.55,24.38 42.93,24.77 42.93,39.24 43.05,39.37 v43.18,39.37 | UART.2 55.88,40.51 54.85,41.54 54.85,44.69 J3.2 | U3.1 57.62,30.82 58.17,31.37 58.17,41.53 v57.79,41.91
PD4/A6/D4  (via drill 0.3 pad 0.64)
  Top 0.203: J3.5 53.34,45.21 52.71,44.58 v43.43,44.58
  Bottom 0.203: U7.25 43.08,21.18 43.82,21.92 43.82,42.8 43.43,43.18 v43.43,44.58
PD5/TXLED  (via drill 0.3 pad 0.64)
  Top 0.203: v39.62,23.75 37.34,26.04 22.86,26.04 21.97,25.15 21.97,21.84 v22.61,21.21
  Bottom 0.203: U7.22 39.33,23.45 v39.62,23.75 | R28.1 v22.61,21.21
PD6/A11/D12  (via drill 0.3 pad 0.64)
  Top 0.203: v44.2,43.81 43.31,43.81 42.55,44.58 v33.66,44.58
  Bottom 0.203: U7.26 43.09,20.68 44.2,21.79 v44.2,43.81 | J4.5 34.93,47.37 MISO.MM MISO.11 v33.66,44.58
PD6/D5
  Bottom 0.203: U7.31 43.33,18.18 46.1,20.95 46.1,31.88 49.78,35.56 49.78,45.09 50.67,45.97 50.67,50.67 J3.6
PD7/A7/D6
  Bottom 0.203: U7.27 43.13,20.18 44.58,21.63 44.58,32.51 48.26,36.2 J3.7
PE6/D7  (via drill 0.3 pad 0.64)
  Top 0.203: v47.12,21.59 47.12,19.05 39.37,11.3 32.39,11.3 29.21,14.48 v29.21,16.76 | v52.07,48.26 48.26,48.26 J3.8
  Bottom 0.203: U7.1 33.19,17.18 32.77,16.76 v29.21,16.76 | v47.12,21.59 47.12,31.62 50.55,35.05 50.55,43.43 52.07,44.96 v52.07,48.26
PF0/A5  (via drill 0.3 pad 0.64)
  Top 0.203: J5.6 61.2,4.84 45.61,4.84 v44.96,4.19
  Bottom 0.203: U7.41 35.83,15.61 36.07,15.37 36.07,13.59 34.93,12.45 | v44.96,4.19 44.96,4.45 41.78,7.62 36.83,7.62 36.07,8.38 36.07,9.91 35.81,10.16 | SCL.MM SCL.00
  Bottom 0.406: SCL.MM 35.81,10.16 | SCL.00 34.93,12.45
PF1/A4  (via drill 0.3 pad 0.64)
  Top 0.203: J5.5 59.05,4.45 46.23,4.45 v45.85,4.06
  Bottom 0.203: U7.40 36.33,15.74 36.45,15.62 36.45,13.84 37.47,12.83 37.47,12.45 | v45.85,4.06 45.85,4.19 42.04,8 39.12,8 38.73,8.38 38.73,9.78 38.35,10.16 | SDA.MM SDA.00
  Bottom 0.406: SDA.MM 38.35,10.16 | SDA.00 37.47,12.45
PF4/A3  (via drill 0.3 pad 0.64)
  Top 0.203: J5.4 58.42,2.67 57.02,4.06 48.26,4.06 v47.24,3.05
  Bottom 0.203: U7.39 36.83,13.97 47.24,3.56 v47.24,3.05
PF5/A2
  Bottom 0.203: U7.38 37.33,13.98 48.77,2.54 48.77,1.65 49.53,0.89 54.23,0.89 J5.3
PF6/A1
  Bottom 0.203: U7.37 37.83,13.99 49.15,2.67 49.15,1.78 49.66,1.27 52.07,1.27 J5.2
PF7/A0
  Bottom 0.203: U7.36 38.33,13.99 49.78,2.54 J5.1
UART_RX  (via drill 0.3 pad 0.64)
  Top 0.203: U2.33 40.01,8.2 51.87,20.07 55.63,20.07 v56.26,20.7
  Bottom 0.203: U3.4 56.68,28.87 55.88,28.07 55.88,21.08 v56.26,20.7
UART_TX  (via drill 0.3 pad 0.64)
  Top 0.203: U2.34 37.47,8.51 37.85,8.89 40.13,8.89 51.69,20.45 54.99,20.45 v55.25,20.7
  Bottom 0.203: U3.5 54.57,28.87 55.5,27.94 55.5,20.95 v55.25,20.7
UCAP
  Bottom 0.203: U7.6 32.64,19.68 32.51,19.56 31.24,19.56 C18.2
USB_DM  (via drill 0.3 pad 0.64)
  Top 0.203: U2.50 17.89,29.73 18.86,28.77 20.13,28.77 20.95,27.94 v20.95,9.53
  Bottom 0.203: J2.DM 12.6,9.78 14.73,9.78 15.37,10.41 D3.2 20.07,10.41 v20.95,9.53
USB_DP  (via drill 0.3 pad 0.64)
  Top 0.203: U2.49 17.39,27.3 17.91,27.3 18.86,28.26 19.88,28.26 20.45,27.69 20.45,9.91 v20.07,9.53
  Bottom 0.203: J2.DP 12.6,9.27 14.73,9.27 15.37,8.64 D3.1 16.89,8.64 arc-90 17.14,8.38 17.14,7.89 arc90 17.4,7.63 17.53,7.63 arc90 17.78,7.89 17.78,8.38 arc-90 18.03,8.64 19.18,8.64 v20.07,9.53

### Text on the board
tPlace: D8 | D7 | D4 | D2 | D1 | D0 | GND | D12 | *D9 | *D6 | *D5 | *D3 | SCL | SDA | AREF | *D13 | *D11 | *D10 | SCL | RX | SDA | TX | VCC | VCC | GND | GND | NC | IO / REF | RST | 3V3 | 5V | GND | GND | VIN | A0 | A1 | A2 | A3 | A4 | A5
bPlace: D13 | SCK | D12 | MISO | D11 | MOSI | Seeeduino Cloud | v1.0 07/16/2014 | by Seeed Studio | VCC | www.seeedstudio.com | MISO | SCK | MOSI | RST | GND | A5 | A4
bNames: U3 | U8 | U5
tValues: Valid combinations: | 3.3V Reg / 8MHz | 5V Reg / 16MHz | Mark back accordingly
